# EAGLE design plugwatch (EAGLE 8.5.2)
AUTHOR: Noah Klugman; REV: B; TITLE: PlugWatch

## Sheet 1 of 4: Headers
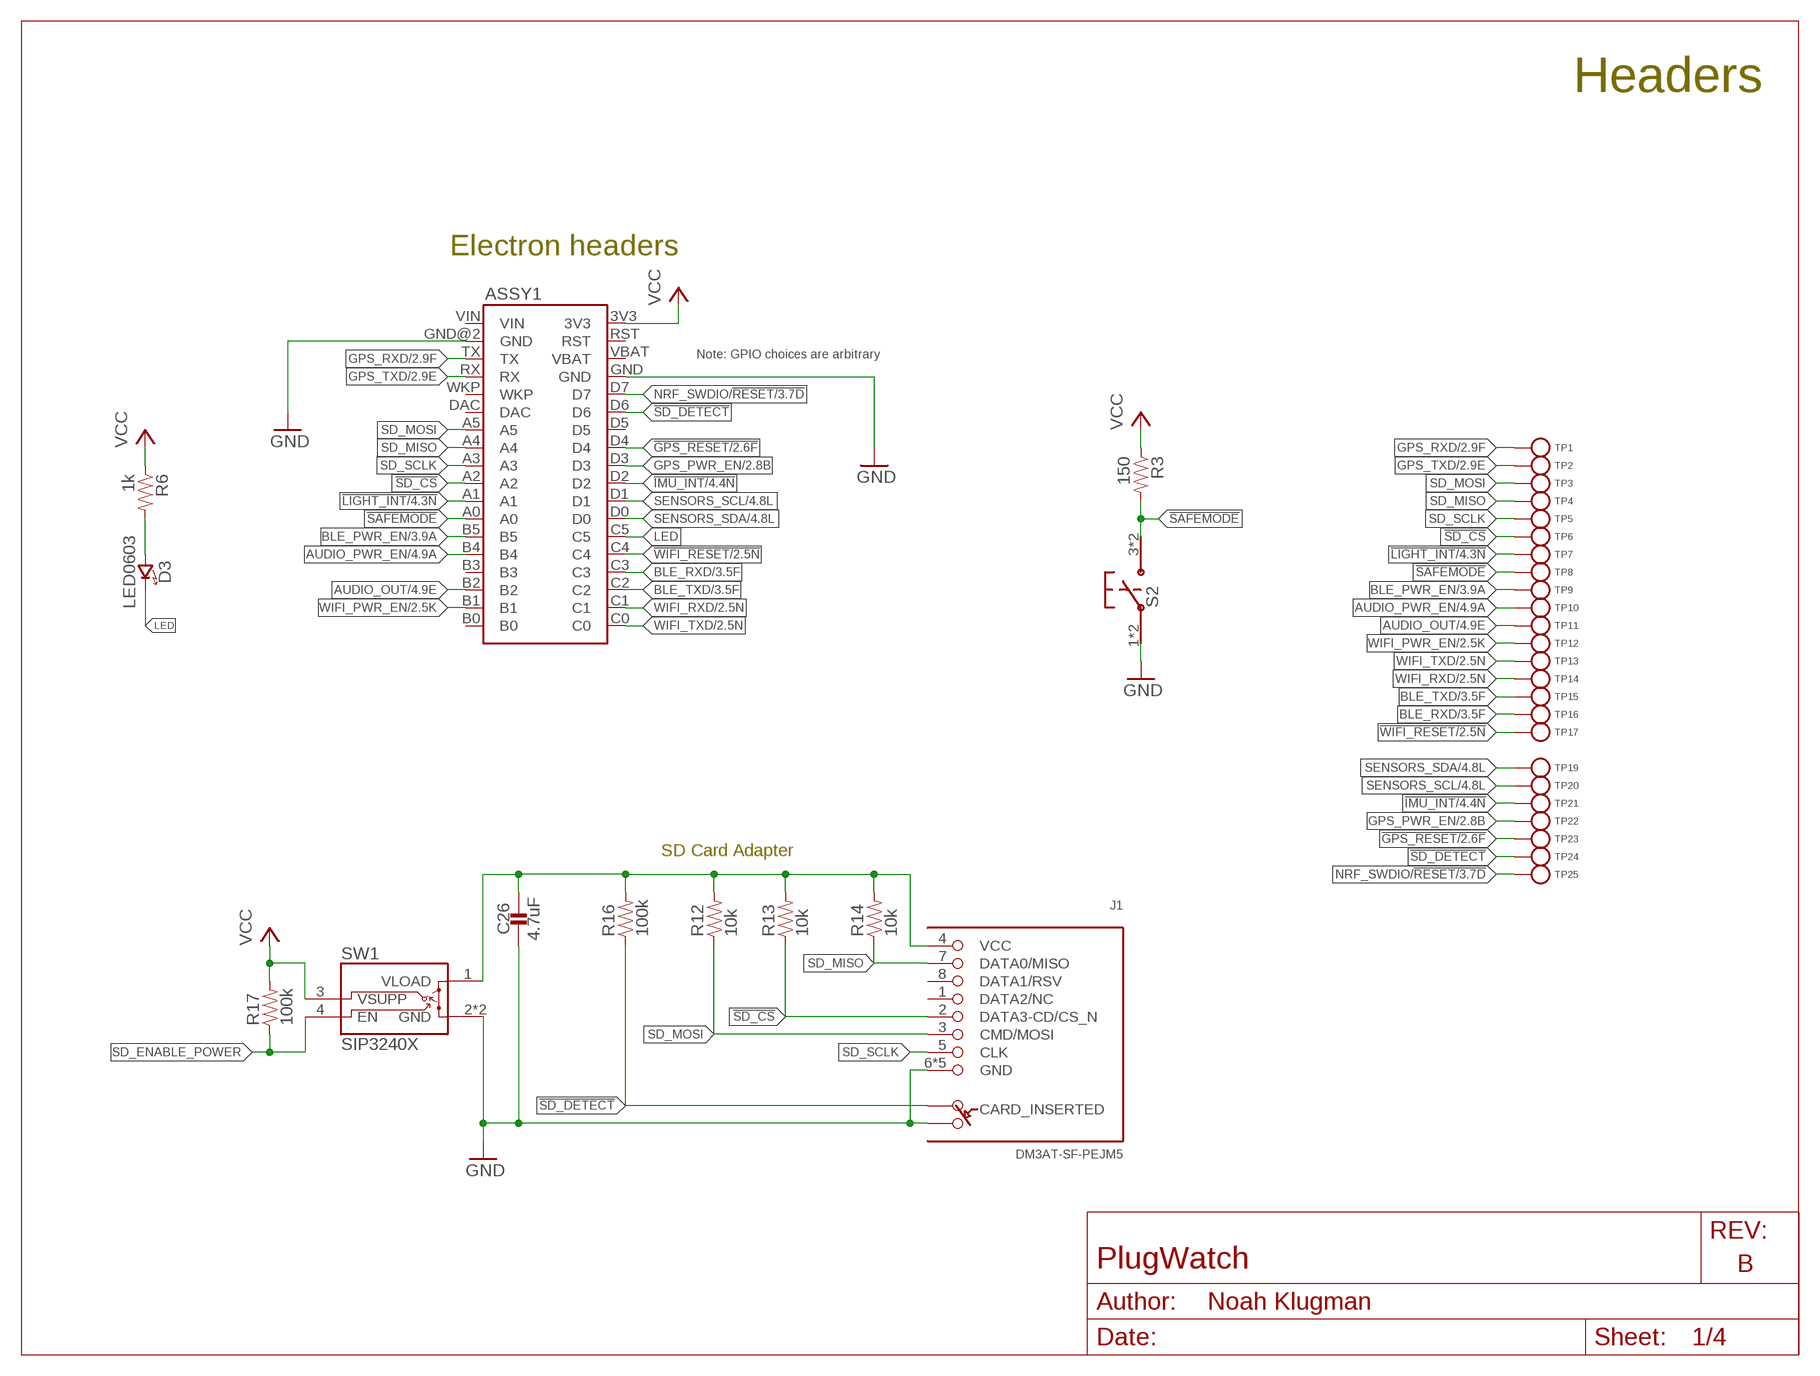
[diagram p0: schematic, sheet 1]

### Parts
ASSY1  ELECTRON  [ELECTRON_SINGLE-ROW]
C26  4.7uF  CAPACITOR0402_CAP  [0402_CAP]
D3  LED0603  [LED-0603]
J1  DM3AT-SF-PEJM5  [DM3AT-SF-PEJM5]
R3  150  RESISTOR0402_RES  [0402_RES]
R6  1k  RESISTOR0402_RES  [0402_RES]
R12  10k  RESISTOR0402_RES  [0402_RES]
R13  10k  RESISTOR0402_RES  [0402_RES]
R14  10k  RESISTOR0402_RES  [0402_RES]
R16  100k  RESISTOR0402_RES  [0402_RES]
R17  100k  RESISTOR0402_RES  [0402_RES]
S2  PTS645SM43SMTR92  [PTS645]
SW1  SIP3240X  [TDFN4]
TP1  TEST_POINT_0.040IN  [TESTPOINT_0.040IN]
TP2  TEST_POINT_0.040IN  [TESTPOINT_0.040IN]
TP3  TEST_POINT_0.040IN  [TESTPOINT_0.040IN]
TP4  TEST_POINT_0.040IN  [TESTPOINT_0.040IN]
TP5  TEST_POINT_0.040IN  [TESTPOINT_0.040IN]
TP6  TEST_POINT_0.040IN  [TESTPOINT_0.040IN]
TP7  TEST_POINT_0.040IN  [TESTPOINT_0.040IN]
TP8  TEST_POINT_0.040IN  [TESTPOINT_0.040IN]
TP9  TEST_POINT_0.040IN  [TESTPOINT_0.040IN]
TP10  TEST_POINT_0.040IN  [TESTPOINT_0.040IN]
TP11  TEST_POINT_0.040IN  [TESTPOINT_0.040IN]
TP12  TEST_POINT_0.040IN  [TESTPOINT_0.040IN]
TP13  TEST_POINT_0.040IN  [TESTPOINT_0.040IN]
TP14  TEST_POINT_0.040IN  [TESTPOINT_0.040IN]
TP15  TEST_POINT_0.040IN  [TESTPOINT_0.040IN]
TP16  TEST_POINT_0.040IN  [TESTPOINT_0.040IN]
TP17  TEST_POINT_0.040IN  [TESTPOINT_0.040IN]
TP19  TEST_POINT_0.040IN  [TESTPOINT_0.040IN]
TP20  TEST_POINT_0.040IN  [TESTPOINT_0.040IN]
TP21  TEST_POINT_0.040IN  [TESTPOINT_0.040IN]
TP22  TEST_POINT_0.040IN  [TESTPOINT_0.040IN]
TP23  TEST_POINT_0.040IN  [TESTPOINT_0.040IN]
TP24  TEST_POINT_0.040IN  [TESTPOINT_0.040IN]
TP25  TEST_POINT_0.040IN  [TESTPOINT_0.040IN]

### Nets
!GPS_RESET: ASSY1.D4 TP23.TESTPOINT ; also sheet 2
!IMU_INT: ASSY1.D2 TP21.TESTPOINT ; also sheet 4
!LIGHT_INT: ASSY1.A1 TP7.TESTPOINT ; also sheet 4
!SAFEMODE: ASSY1.A0 R3.2 S2.3 S2.4 TP8.TESTPOINT
!SD_CS: ASSY1.A2 J1.2(DATA3-CD/CS_N) R13.1 TP6.TESTPOINT
!SD_DETECT: ASSY1.D6 J1.A R16.1 TP24.TESTPOINT
!WIFI_RESET: ASSY1.C4 TP17.TESTPOINT ; also sheet 2
AUDIO_OUT: ASSY1.B2 TP11.TESTPOINT ; also sheet 4
AUDIO_PWR_EN: ASSY1.B4 TP10.TESTPOINT ; also sheet 4
BLE_PWR_EN: ASSY1.B5 TP9.TESTPOINT ; also sheet 3
BLE_RXD: ASSY1.C3 TP16.TESTPOINT ; also sheet 3
BLE_TXD: ASSY1.C2 TP15.TESTPOINT ; also sheet 3
GND: ASSY1.GND ASSY1.GND@2(GND) C26.2 J1.6(GND) J1.B J1.MOUNT0(GND) J1.MOUNT1(GND) J1.MOUNT2(GND) J1.MOUNT3(GND) S2.1 S2.2 SW1.2(GND) SW1.PAD(GND) ; also sheet 2,3,4
GPS_PWR_EN: ASSY1.D3 TP22.TESTPOINT ; also sheet 2
GPS_RXD: ASSY1.TX TP1.TESTPOINT ; also sheet 2
GPS_TXD: ASSY1.RX TP2.TESTPOINT ; also sheet 2
LED: ASSY1.C5 D3.C(CATHODE)
N$3: D3.A(ANODE) R6.2
N$18: C26.1 J1.4(VCC) R12.2 R13.2 R14.2 R16.2 SW1.1(VLOAD)
NRF_SWDIO/!RESET: ASSY1.D7 TP25.TESTPOINT ; also sheet 3
SD_ENABLE_POWER: R17.1 SW1.4(EN)
SD_MISO: ASSY1.A4 J1.7(DATA0/MISO) R14.1 TP4.TESTPOINT
SD_MOSI: ASSY1.A5 J1.3(CMD/MOSI) R12.1 TP3.TESTPOINT
SD_SCLK: ASSY1.A3 J1.5(CLK) TP5.TESTPOINT
SENSORS_SCL: ASSY1.D1 TP20.TESTPOINT ; also sheet 4
SENSORS_SDA: ASSY1.D0 TP19.TESTPOINT ; also sheet 4
VCC: ASSY1.3V3 R3.1 R6.1 R17.2 SW1.3(VSUPP) ; also sheet 2,3,4
WIFI_PWR_EN: ASSY1.B1 TP12.TESTPOINT ; also sheet 2
WIFI_RXD: ASSY1.C1 TP14.TESTPOINT ; also sheet 2
WIFI_TXD: ASSY1.C0 TP13.TESTPOINT ; also sheet 2
Unconnected: ASSY1.B0 ASSY1.B3 ASSY1.D5 ASSY1.DAC ASSY1.RST ASSY1.VBAT ASSY1.WKP J1.1(DATA2/NC) J1.8(DATA1/RSV)

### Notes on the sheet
- Headers
- Electron headers
- Note: GPIO choices are arbitrary
- SD Card Adapter

## Sheet 2 of 4: GPS and WiFi Radios
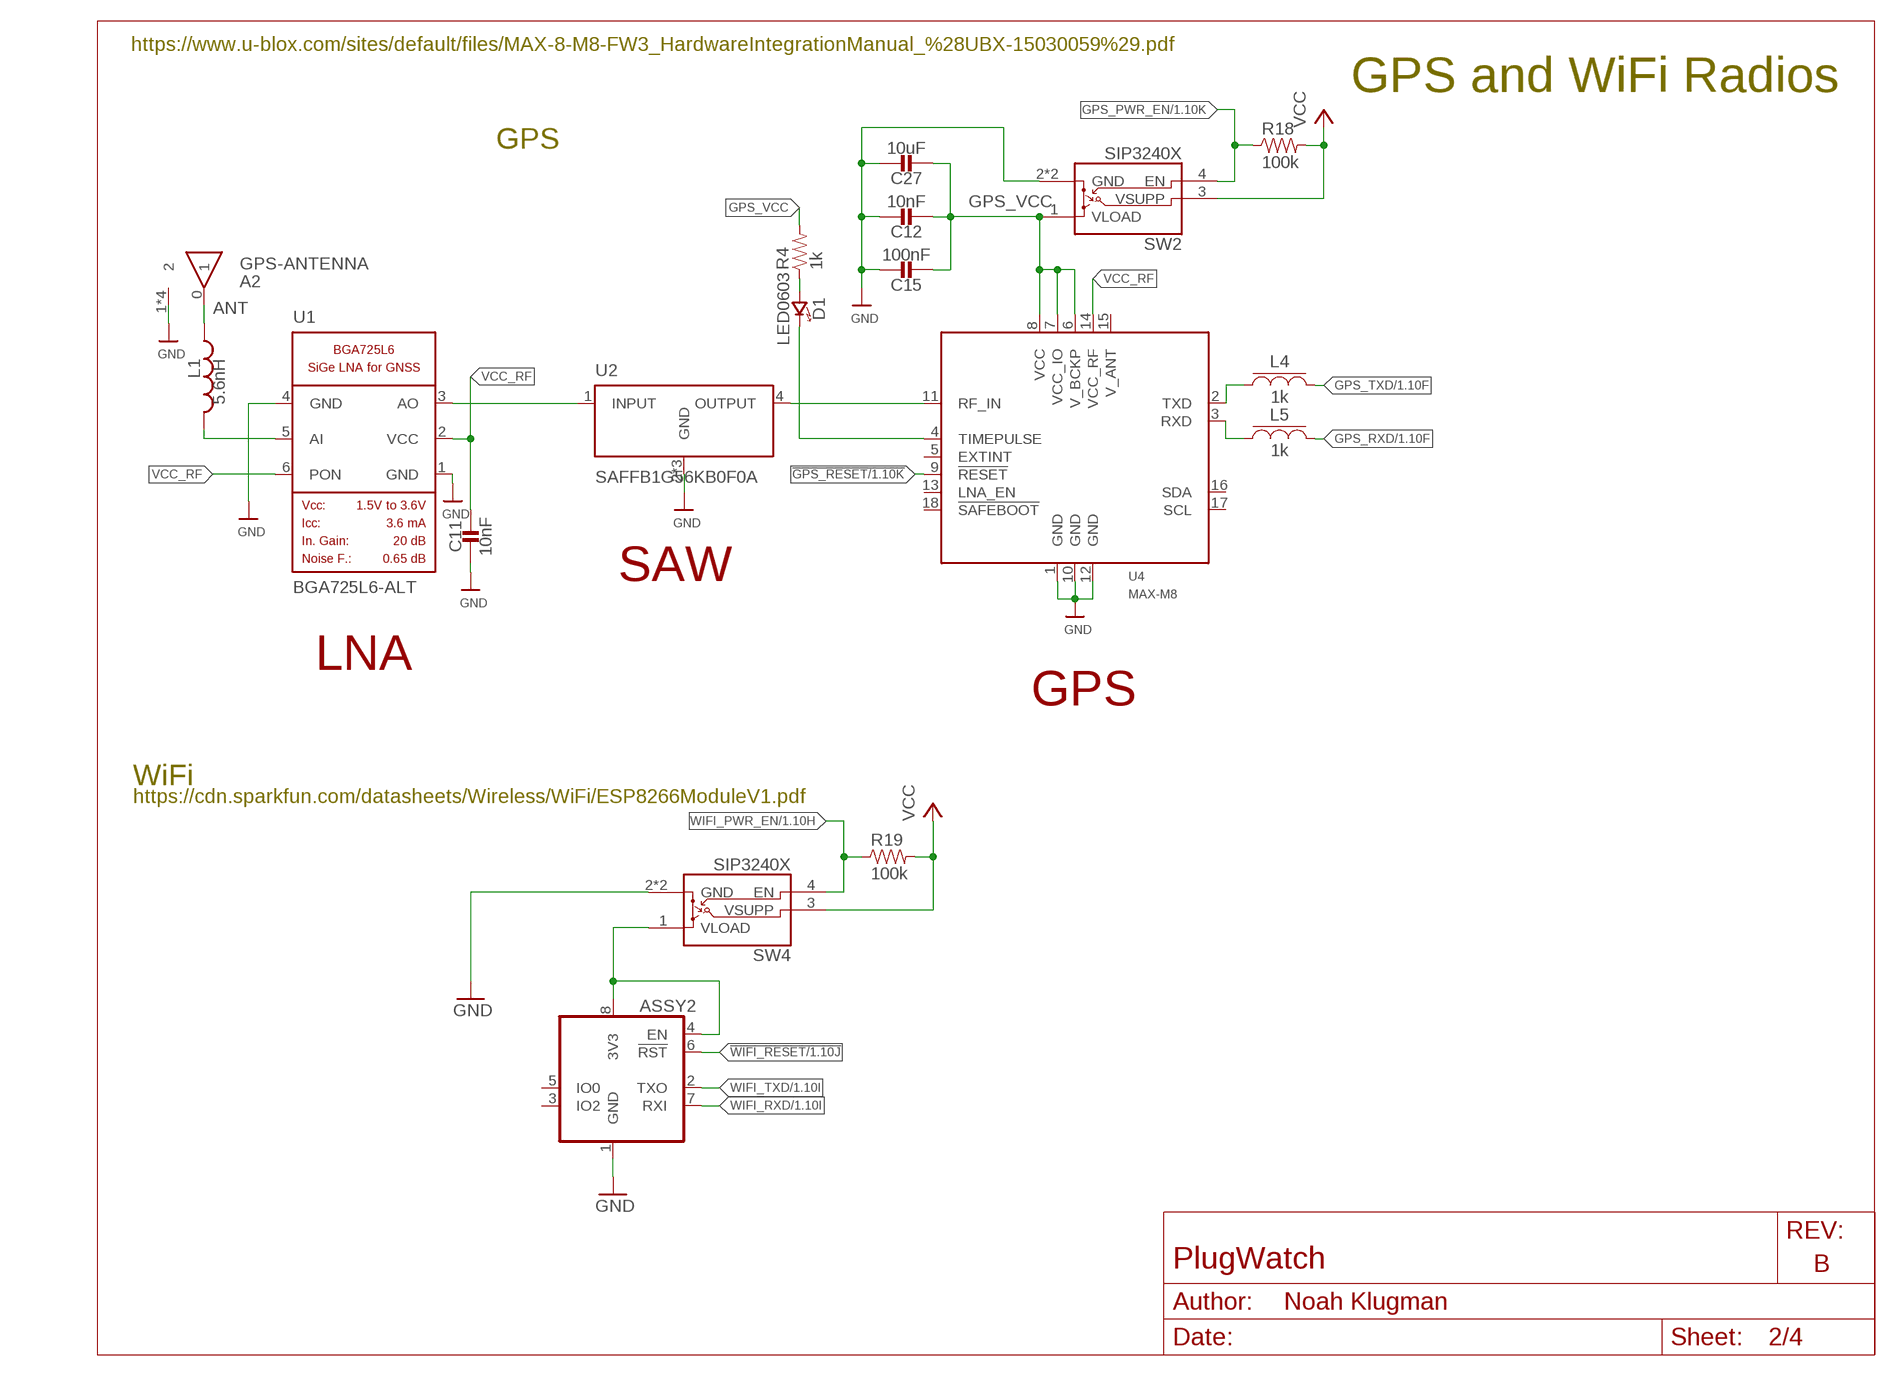
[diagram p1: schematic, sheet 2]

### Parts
A2  GPS-ANTENNA  [ANT1818B00BT1516S]
ASSY2  WRL-13678  [WRL-13678]
C11  10nF  CAPACITOR0402_CAP  [0402_CAP]
C12  10nF  CAPACITOR0402_CAP  [0402_CAP]
C15  100nF  CAPACITOR0402_CAP  [0402_CAP]
C27  10uF  CAPACITOR0402_CAP  [0402_CAP]
D1  LED0603  [LED-0603]
L1  5.6nH  INDUCTOR0402  [0402_CAP]
L4  1k  FERRITE_BEAD0402  [0402_CAP]
L5  1k  FERRITE_BEAD0402  [0402_CAP]
R4  1k  RESISTOR0402_RES  [0402_RES]
R18  100k  RESISTOR0402_RES  [0402_RES]
R19  100k  RESISTOR0402_RES  [0402_RES]
SW2  SIP3240X  [TDFN4]
SW4  SIP3240X  [TDFN4]
U1  BGA725L6-ALT  [LNA-TSLP-6-2-ALT]
U2  SAFFB1G56KB0F0A  FILTERS  [QCS5I]
U4  MAX-M8  [MAX-M8]

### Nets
!GPS_RESET: U4.9(!RESET) ; also sheet 1
!WIFI_RESET: ASSY2.6(!RST) ; also sheet 1
ANT: A2.0 L1.2
GND: A2.1 A2.2 A2.3 A2.4 ASSY2.1(GND) C11.1 C12.1 C15.1 C27.1 SW2.2(GND) SW2.PAD(GND) SW4.2(GND) SW4.PAD(GND) U1.1(GND) U1.4(GND) U2.2(GND) U2.3(GND) U2.5(GND) U4.1(GND) U4.10(GND) U4.12(GND) ; also sheet 1,3,4
GPS_PWR_EN: R18.1 SW2.4(EN) ; also sheet 1
GPS_RF_IN: U2.4(OUTPUT) U4.11(RF_IN)
GPS_RXD: L5.2 ; also sheet 1
GPS_TXD: L4.2 ; also sheet 1
GPS_VCC: C12.2 C15.2 C27.2 R4.2 SW2.1(VLOAD) U4.6(V_BCKP) U4.7(VCC_IO) U4.8(VCC)
LNA_IN: L1.1 U1.5(AI)
LNA_OUT: U1.3(AO) U2.1(INPUT)
N$1: D1.A(ANODE) R4.1
N$2: D1.C(CATHODE) U4.4(TIMEPULSE)
N$14: ASSY2.4(EN) ASSY2.8(3V3) SW4.1(VLOAD)
N$40: L4.1 U4.2(TXD)
N$41: L5.1 U4.3(RXD)
VCC: R18.2 R19.2 SW2.3(VSUPP) SW4.3(VSUPP) ; also sheet 1,3,4
VCC_RF: C11.2 U1.2(VCC) U1.6(PON) U4.14(VCC_RF)
WIFI_PWR_EN: R19.1 SW4.4(EN) ; also sheet 1
WIFI_RXD: ASSY2.7(RXI) ; also sheet 1
WIFI_TXD: ASSY2.2(TXO) ; also sheet 1
Unconnected: ASSY2.3(IO2) ASSY2.5(IO0) U4.5(EXTINT) U4.13(LNA_EN) U4.15(V_ANT) U4.16(SDA) U4.17(SCL) U4.18(!SAFEBOOT)

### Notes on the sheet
- https://www.u-blox.com/sites/default/files/MAX-8-M8-FW3_HardwareIntegrationManual_%28UBX-15030059%29.pdf
- GPS and WiFi Radios
- GPS
- SAW
- LNA
- GPS
- WiFi
- https://cdn.sparkfun.com/datasheets/Wireless/WiFi/ESP8266ModuleV1.pdf

## Sheet 3 of 4: BLE Radio
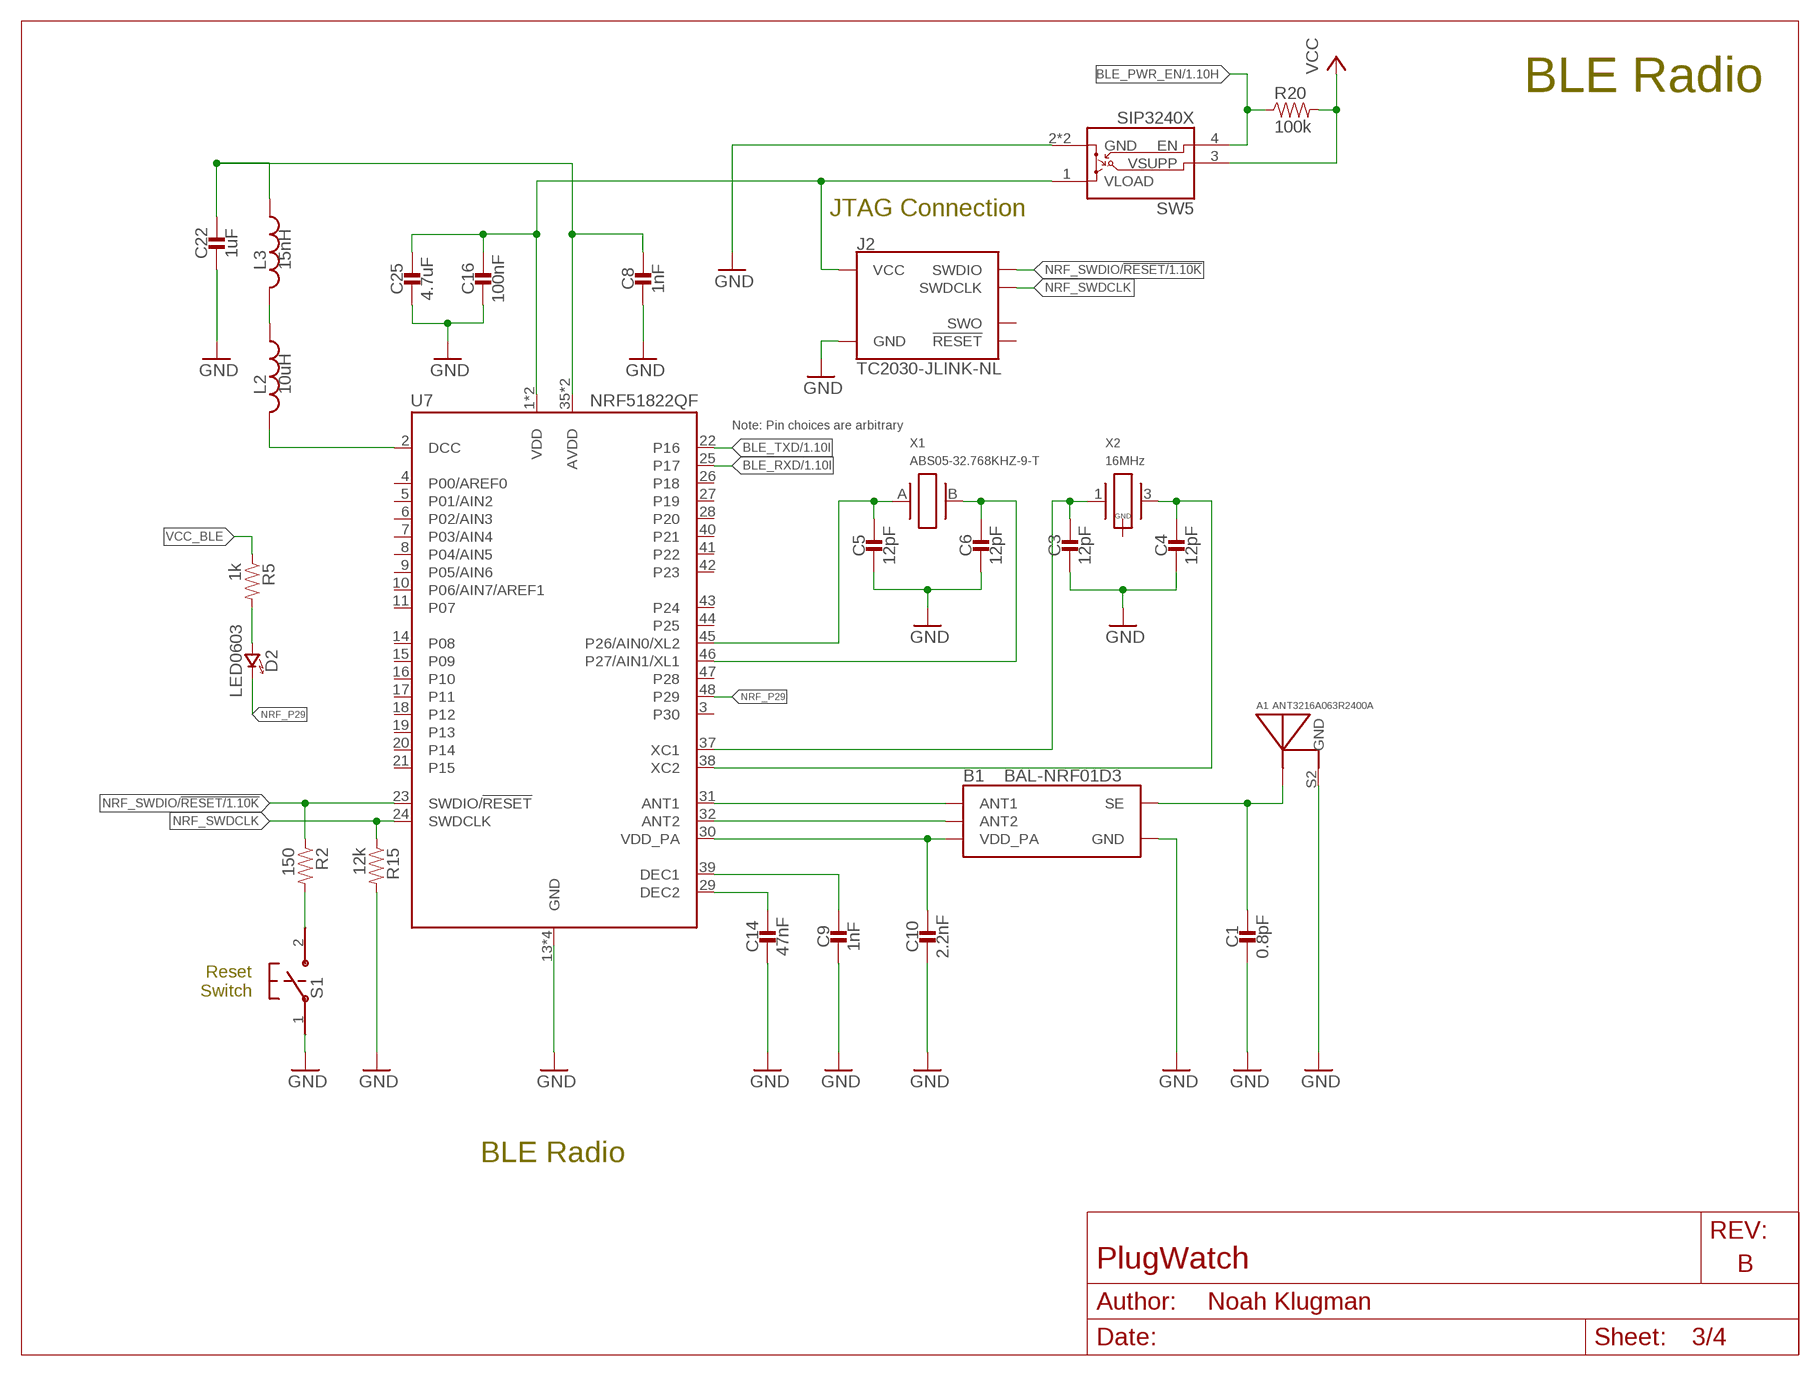
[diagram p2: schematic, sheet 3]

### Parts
A1  ANT3216A063R2400A  [ANT3216A063R2400A]
B1  BAL-NRF01D3  [BAL-NRF01D3]
C1  0.8pF  CAPACITOR0402_CAP  [0402_CAP]
C3  12pF  CAPACITOR0402_CAP  [0402_CAP]
C4  12pF  CAPACITOR0402_CAP  [0402_CAP]
C5  12pF  CAPACITOR0402_CAP  [0402_CAP]
C6  12pF  CAPACITOR0402_CAP  [0402_CAP]
C8  1nF  CAPACITOR0402_CAP  [0402_CAP]
C9  1nF  CAPACITOR0402_CAP  [0402_CAP]
C10  2.2nF  CAPACITOR0402_CAP  [0402_CAP]
C14  47nF  CAPACITOR0402_CAP  [0402_CAP]
C16  100nF  CAPACITOR0402_CAP  [0402_CAP]
C22  1uF  CAPACITOR0402_CAP  [0402_CAP]
C25  4.7uF  CAPACITOR0402_CAP  [0402_CAP]
D2  LED0603  [LED-0603]
J2  TC2030-JLINK-NL  [TC2030-IDC-NL]
L2  10uH  INDUCTOR0603  [0603_CAP]
L3  15nH  INDUCTOR0402  [0402_CAP]
R2  150  RESISTOR0402_RES  [0402_RES]
R5  1k  RESISTOR0402_RES  [0402_RES]
R15  12k  RESISTOR0402_RES  [0402_RES]
R20  100k  RESISTOR0402_RES  [0402_RES]
S1  B3U-1000P  [B3U-1000P]
SW5  SIP3240X  [TDFN4]
U7  NRF51822QF  [QFN-48-6MM]
X1  ABS05-32.768KHZ-9-T  [ABS05]
X2  16MHz  TXC-8Y  [TXC-8Y]

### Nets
AVDD1: C8.1 C22.1 L3.1 U7.35(AVDD) U7.36(AVDD)
BLE_PWR_EN: R20.1 SW5.4(EN) ; also sheet 1
BLE_RXD: U7.25(P17) ; also sheet 1
BLE_TXD: U7.22(P16) ; also sheet 1
DCC1: L2.2 U7.2(DCC)
GND: A1.S2(GND) B1.GND C1.2 C3.2 C4.2 C5.2 C6.2 C8.2 C9.2 C10.2 C14.2 C16.2 C22.2 C25.2 J2.5(GND) R15.2 S1.1 SW5.2(GND) SW5.PAD(GND) U7.13(GND) U7.33(GND) U7.34(GND) U7.GND ; also sheet 1,2,4
N$10: B1.ANT1 U7.31(ANT1)
N$12: B1.ANT2 U7.32(ANT2)
N$13: A1.S1(ANTENNA) B1.SE C1.1
N$15: L2.1 L3.2
N$20: C3.1 U7.37(XC1) X2.1
N$21: C4.1 U7.38(XC2) X2.3
N$22: C9.1 U7.39(DEC1)
N$24: C14.1 U7.29(DEC2)
N$25: D2.A(ANODE) R5.2
N$26: R2.2 S1.2
NRF_A2: C6.1 U7.46(P27/AIN1/XL1) X1.B
NRF_A3: C5.1 U7.45(P26/AIN0/XL2) X1.A
NRF_P29: D2.C(CATHODE) U7.48(P29)
NRF_SWDCLK: J2.4(SWDCLK) R15.1 U7.24(SWDCLK)
NRF_SWDIO/!RESET: J2.2(SWDIO) R2.1 U7.23(SWDIO/!RESET) ; also sheet 1
VCC: R20.2 SW5.3(VSUPP) ; also sheet 1,2,4
VCC_BLE: C16.1 C25.1 J2.1(VCC) R5.1 SW5.1(VLOAD) U7.1(VDD) U7.12(VDD)
VDD_PA1: B1.VCC(VDD_PA) C10.1 U7.30(VDD_PA)
Unconnected: J2.3(!RESET) J2.6(SWO) U7.3(P30) U7.4(P00/AREF0) U7.5(P01/AIN2) U7.6(P02/AIN3) U7.7(P03/AIN4) U7.8(P04/AIN5) U7.9(P05/AIN6) U7.10(P06/AIN7/AREF1) U7.11(P07) U7.14(P08) U7.15(P09) U7.16(P10) U7.17(P11) U7.18(P12) U7.19(P13) U7.20(P14) U7.21(P15) U7.26(P18) U7.27(P19) U7.28(P20) U7.40(P21) U7.41(P22) U7.42(P23) U7.43(P24) U7.44(P25) U7.47(P28) X2.2(GND) X2.4(GND)

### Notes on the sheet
- BLE Radio
- JTAG Connection
- Note: Pin choices are arbitrary
- Reset
  Switch
- BLE Radio

## Sheet 4 of 4: Sensors
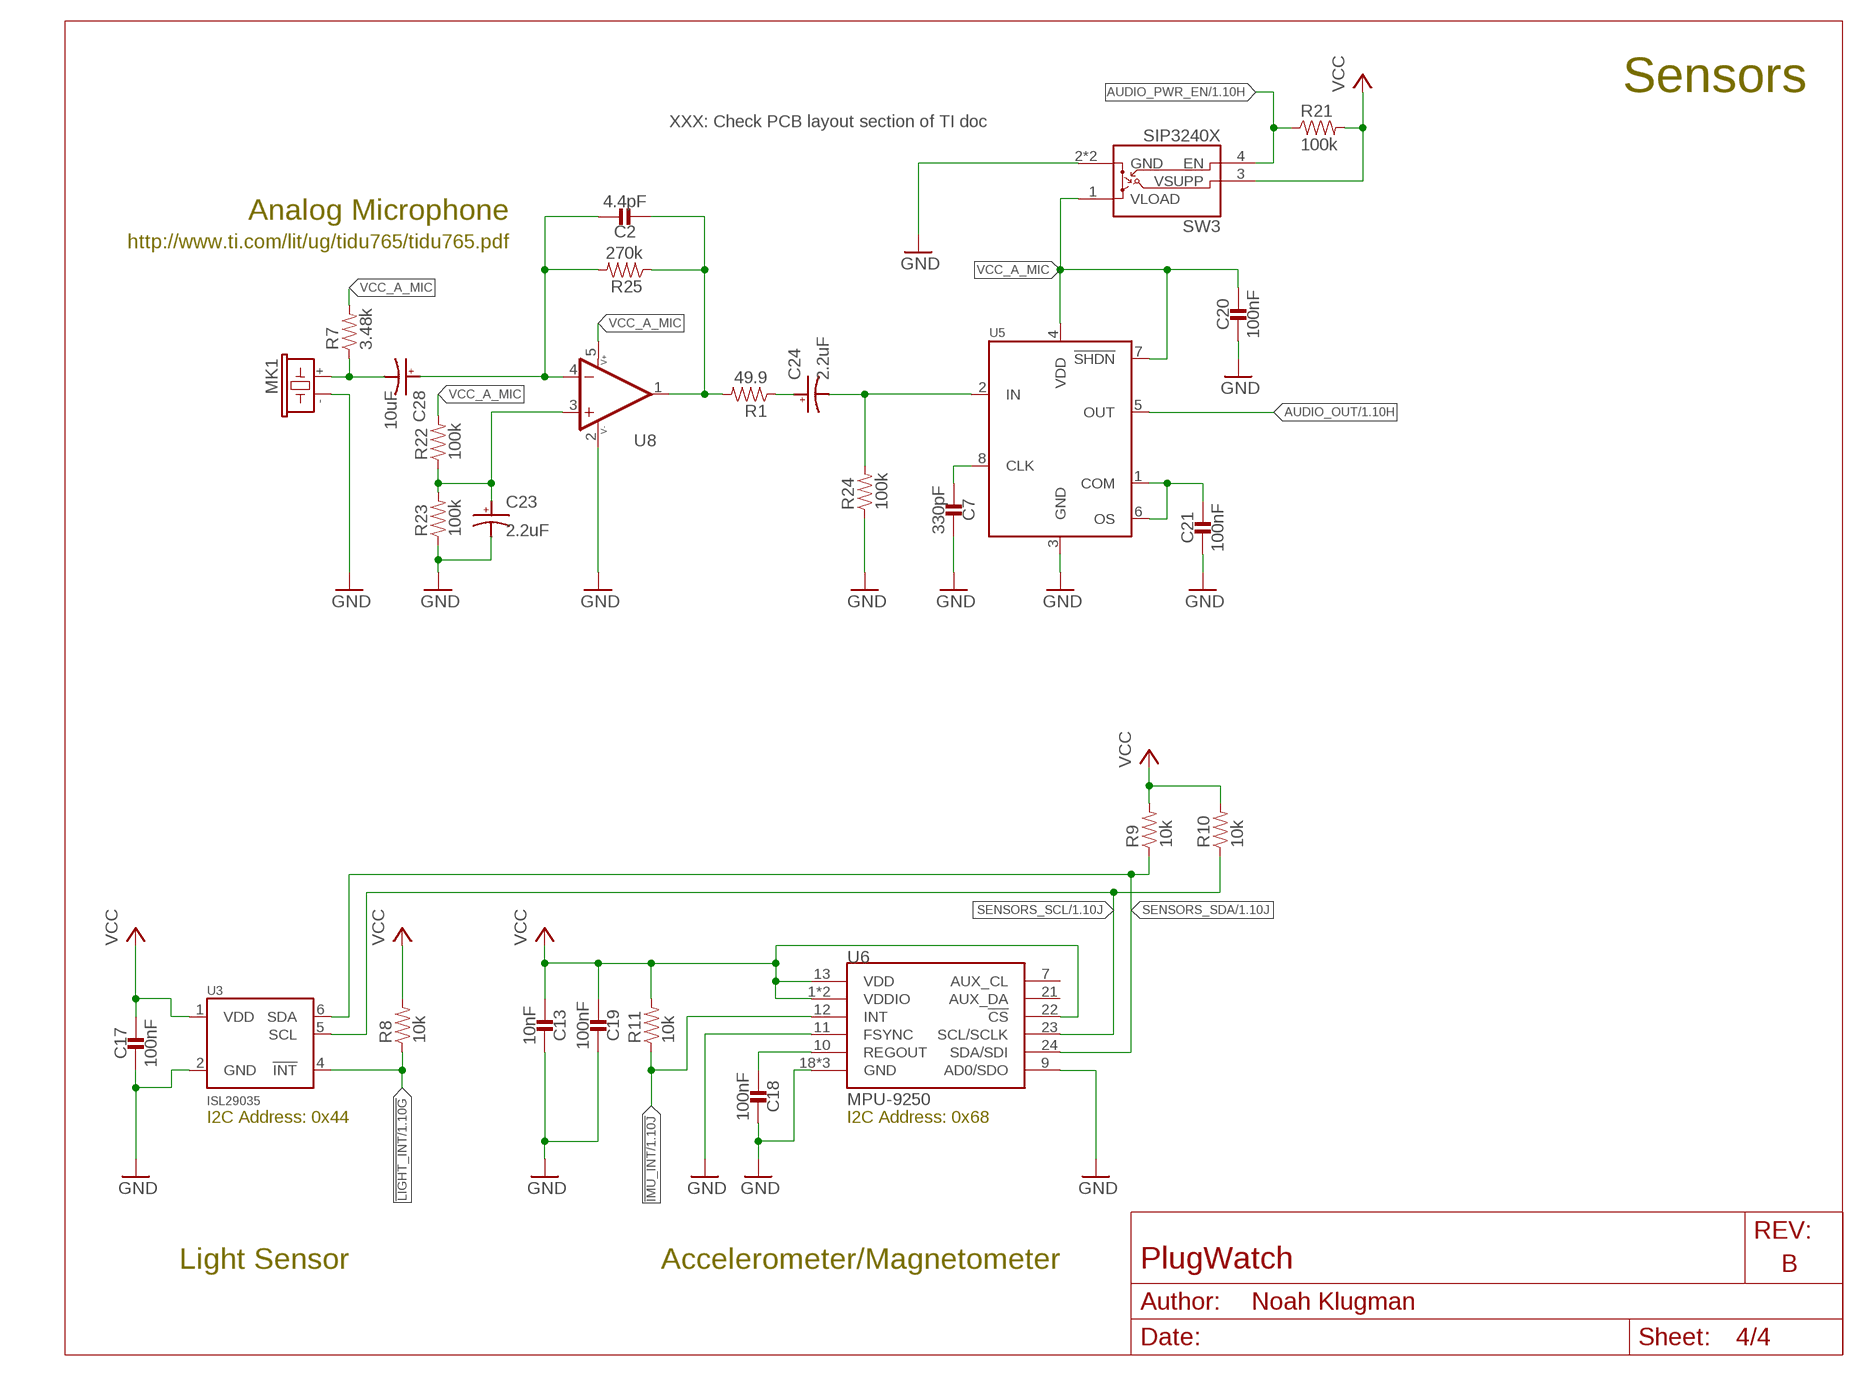
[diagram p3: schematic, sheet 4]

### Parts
C2  4.4pF  CAPACITOR0603_CAP  [0603_CAP]
C7  330pF  CAPACITOR0402_CAP  [0402_CAP]
C13  10nF  CAPACITOR0402_CAP  [0402_CAP]
C17  100nF  CAPACITOR0402_CAP  [0402_CAP]
C18  100nF  CAPACITOR0402_CAP  [0402_CAP]
C19  100nF  CAPACITOR0402_CAP  [0402_CAP]
C20  100nF  CAPACITOR0402_CAP  [0402_CAP]
C21  100nF  CAPACITOR0402_CAP  [0402_CAP]
C23  2.2uF  CAP_POL1206  [1206]
C24  2.2uF  CAP_POL1206  [1206]
C28  10uF  CAP_POL1206  [1206]
MK1  AOM-4546P-R  [MIC_AOM-4546P-R]
R1  49.9  RESISTOR0603_RES  [0603-RES]
R7  3.48k  RESISTOR0603_RES  [0603-RES]
R8  10k  RESISTOR0402_RES  [0402_RES]
R9  10k  RESISTOR0402_RES  [0402_RES]
R10  10k  RESISTOR0402_RES  [0402_RES]
R11  10k  RESISTOR0402_RES  [0402_RES]
R21  100k  RESISTOR0402_RES  [0402_RES]
R22  100k  RESISTOR0603_RES  [0603-RES]
R23  100k  RESISTOR0603_RES  [0603-RES]
R24  100k  RESISTOR0603_RES  [0603-RES]
R25  270k  RESISTOR0603_RES  [0603-RES]
SW3  SIP3240X  [TDFN4]
U3  ISL29035  [ODFN-6-1.5MMX1.6MM]
U5  MAX740XESA  [SOIC-8]
U6  MPU-9250  [QFN24_PAD]
U8  OPA322AIDBVT  [SOT23-5]

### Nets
!IMU_INT: R11.1 U6.12(INT) ; also sheet 1
!LIGHT_INT: R8.1 U3.4(!INT) ; also sheet 1
-AMP: C2.1 C28.2(CATHODE) R25.2 U8.4(-IN)
A_MIC_OUT: C24.1(ANODE) R24.2 U5.2(IN)
AUDIO_OUT: U5.5(OUT) ; also sheet 1
AUDIO_PWR_EN: R21.1 SW3.4(EN) ; also sheet 1
GND: C7.1 C13.2 C17.2 C18.2 C19.2 C20.2 C21.2 C23.1(ANODE) MK1.TERM- R23.1 R24.1 SW3.2(GND) SW3.PAD(GND) U3.2(GND) U5.3(GND) U6.9(AD0/SDO) U6.11(FSYNC) U6.18(GND) U6.20(GND) U6.CENTER(GND) U8.2(V-) ; also sheet 1,2,3
N$4: C28.1(ANODE) MK1.TERM+ R7.1
N$5: C2.2 R1.2 R25.1 U8.1(OUT)
N$6: C7.2 U5.8(CLK)
N$7: C24.2(CATHODE) R1.1
N$9: C23.2(CATHODE) R22.1 R23.2 U8.3(+IN)
N$11: C21.1 U5.1(COM) U5.6(OS)
REGOUT: C18.1 U6.10(REGOUT)
SENSORS_SCL: R10.1 U3.5(SCL) U6.23(SCL/SCLK) ; also sheet 1
SENSORS_SDA: R9.1 U3.6(SDA) U6.24(SDA/SDI) ; also sheet 1
VCC: C13.1 C17.1 C19.1 R8.2 R9.2 R10.2 R11.2 R21.2 SW3.3(VSUPP) U3.1(VDD) U6.1(VDDIO) U6.8(VDDIO) U6.13(VDD) U6.22(!CS) ; also sheet 1,2,3
VCC_A_MIC: C20.1 R7.2 R22.2 SW3.1(VLOAD) U5.4(VDD) U5.7(!SHDN) U8.5(V+)
Unconnected: U6.7(AUX_CL) U6.21(AUX_DA)

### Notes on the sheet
- Sensors
- XXX: Check PCB layout section of TI doc
- Analog Microphone
- http://www.ti.com/lit/ug/tidu765/tidu765.pdf
- I2C Address: 0x44 | I2C Address: 0x68
- Light Sensor | Accelerometer/Magnetometer

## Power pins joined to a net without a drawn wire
VIN: ASSY1.VIN

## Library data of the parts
A1 = chips:ANT3216A063R2400A: Yageo 2.4GHz; DIGIKEY: 311-1542-1-ND; MANUFACTURER: YAGEO; MPN: ANT3216A063R2400A
A2 = antenna:GPS-ANTENNA; DIGIKEY: 311-1531-ND
ASSY1 = electron:ELECTRON; DIGIKEY: S7051-ND,S7051-ND
ASSY2 = chips:WRL-13678: ESP8266 WiFi Module https://www.mouser.com/ds/2/813/ESP8266ModuleV1-1095236.pdf; DIGIKEY: 1568-1235-ND
B1 = chips:BAL-NRF01D3: 50 ohm nominal input / conjugate match balun to nRF51422-QFAA, nRF24LE1, nRF51822-QFAA/AB, with integrated harmonic filter; DIGIKEY: 497-13637-1-ND; MANUFACTURER: STMicroelectronics; MOUSER: 511-BAL-NRF01D3; MPN: BAL-NRF01D3
C1 = passives:CAPACITOR: 0402 Capacitor; DIGIKEY: 490-6269-1-ND
C2 = passives:CAPACITOR: 0402 Capacitor; DIGIKEY: 399-16187-1-ND
C3-C6 = passives:CAPACITOR: 0402 Capacitor; DIGIKEY: 490-6197-1-ND
C7 = passives:CAPACITOR: 0402 Capacitor; DIGIKEY: 490-6233-1-ND
C8 C9 = passives:CAPACITOR: 0402 Capacitor; DIGIKEY: 490-6366-1-ND
C10 = passives:CAPACITOR: 0402 Capacitor; DIGIKEY: 490-5419-1-ND
C11-C13 = passives:CAPACITOR: 0402 Capacitor; DIGIKEY: 490-7763-1-ND
C14 = passives:CAPACITOR: 0402 Capacitor; DIGIKEY: 490-11420-1-ND
C15-C21 = passives:CAPACITOR: 0402 Capacitor; DIGIKEY: 490-10777-1-ND
C22 = passives:CAPACITOR: 0402 Capacitor; DIGIKEY: 490-14457-1-ND
C23 C24 = passives:CAP_POL; DIGIKEY: 718-1131-1-ND
C25 C26 = passives:CAPACITOR: 0402 Capacitor; DIGIKEY: 445-5947-1-ND
C27 = passives:CAPACITOR: 0402 Capacitor; DIGIKEY: 490-8316-1-ND
C28 = passives:CAP_POL; DIGIKEY: 478-8481-1-ND
D1-D3 = leds:LED: LED; DIGIKEY: 160-1837-6-ND
J1 = connector:DM3AT-SF-PEJM5: CONN MICRO SD R/A PUSH-PUSH SMD; DIGIKEY: HR1964CT-ND
J2 = connector:TC2030-JLINK
L1 = passives:INDUCTOR: A very specific inductor; DIGIKEY: 490-11766-1-ND
L2 = passives:INDUCTOR: A very specific inductor; DIGIKEY: 490-4025-1-ND
L3 = passives:INDUCTOR: A very specific inductor; DIGIKEY: 587-1521-1-ND
L4 L5 = passives:FERRITE_BEAD; DIGIKEY: 490-4003-1-ND
MK1 = microphones:AOM-4546P-R: Electret microphone; DIGIKEY: 668-1224-ND
R1 = passives:RESISTOR: Resistor; DIGIKEY: 541-3003-1-ND
R2 R3 = passives:RESISTOR: Resistor; DIGIKEY: RMCF0402FT150RCT-ND
R4-R6 = passives:RESISTOR: Resistor; DIGIKEY: RMCF0402FT1K00CT-ND
R7 = passives:RESISTOR: Resistor; DIGIKEY: 541-3.48KHCT-ND
R8-R14 = passives:RESISTOR: Resistor; DIGIKEY: RMCF0402FT10K0CT-ND
R15 = passives:RESISTOR: Resistor; DIGIKEY: RMCF0402FT12K0CT-ND
R16-R21 = passives:RESISTOR: Resistor; DIGIKEY: 1276-3432-1-ND
R22-R24 = passives:RESISTOR: Resistor; DIGIKEY: 541-2972-1-ND
R25 = passives:RESISTOR: Resistor; DIGIKEY: 541-270KHCT-ND
S1 = switches:B3U: Switch; DIGIKEY: SW1020CT-ND; MANUFACTURER: Omron; MPN: B3U-1000P
S2 = switches:PTS645SM43SMTR92: Tactile Switch SPST-NO Top Actuated Surface Mount; DIGIKEY: CKN9112CT-ND
SW1-SW5 = signpost:SIP3240X: High power (2.4 A) high-side switch; DIGIKEY: SIP32402ADNP-T1GE4CT-ND
TP1-TP17 TP19-TP25 = headers:TEST_POINT_0.040IN: 0.040in Test Point; DIGIKEY: 5001K-ND
U1 = Particle:BGA725L6; DIGIKEY: BGA725L6E6327FTSA1CT-ND
U2 = Particle:FILTERS; ABACUS_TECHNOLOGIES: SAFFB1G56KB0F0A
U3 = chips:ISL29035: Optical Sensor Ambient 550nm I2C; DIGIKEY: ISL29035IROZ-T7CT-ND; MPN: ISL29035IROZ-T7
U4 = u-blox:MAX-M8; DIGIKEY: 672-1003-1-ND
U5 = chips:MAX740X; ROCHESTER_ELECTRONICS: MAX7405ESA
U6 = Testing:MPU-9250: NC pin 19. 2-6 & 14-17 not internally connected. May be used for PCB trace routing.; DIGIKEY: 1428-1019-1-ND; PROD_ID: IC-13192
U7 = chips:NRF51822: Multiprotocol Bluetooth® 4.0 low energy/2.4 GHz RF SoC; DIGIKEY: 1490-1049-1-ND; MANUFACTURER: Nordic Semi; MOUSER: 949-NRF51822-QFAC-R7; MPN: NRF51822-QFAC-R7
U8 = opamps:OPA322; DIGIKEY: 296-29511-1-ND
X1 = crystals:ABS05-32.768KHZ: 32.768kHz Crystal; DIGIKEY: 535-11897-1-ND
X2 = crystals:TXC-8Y: 2mmx1.6mm SMD Crystal; DIGIKEY: 887-2003-1-ND

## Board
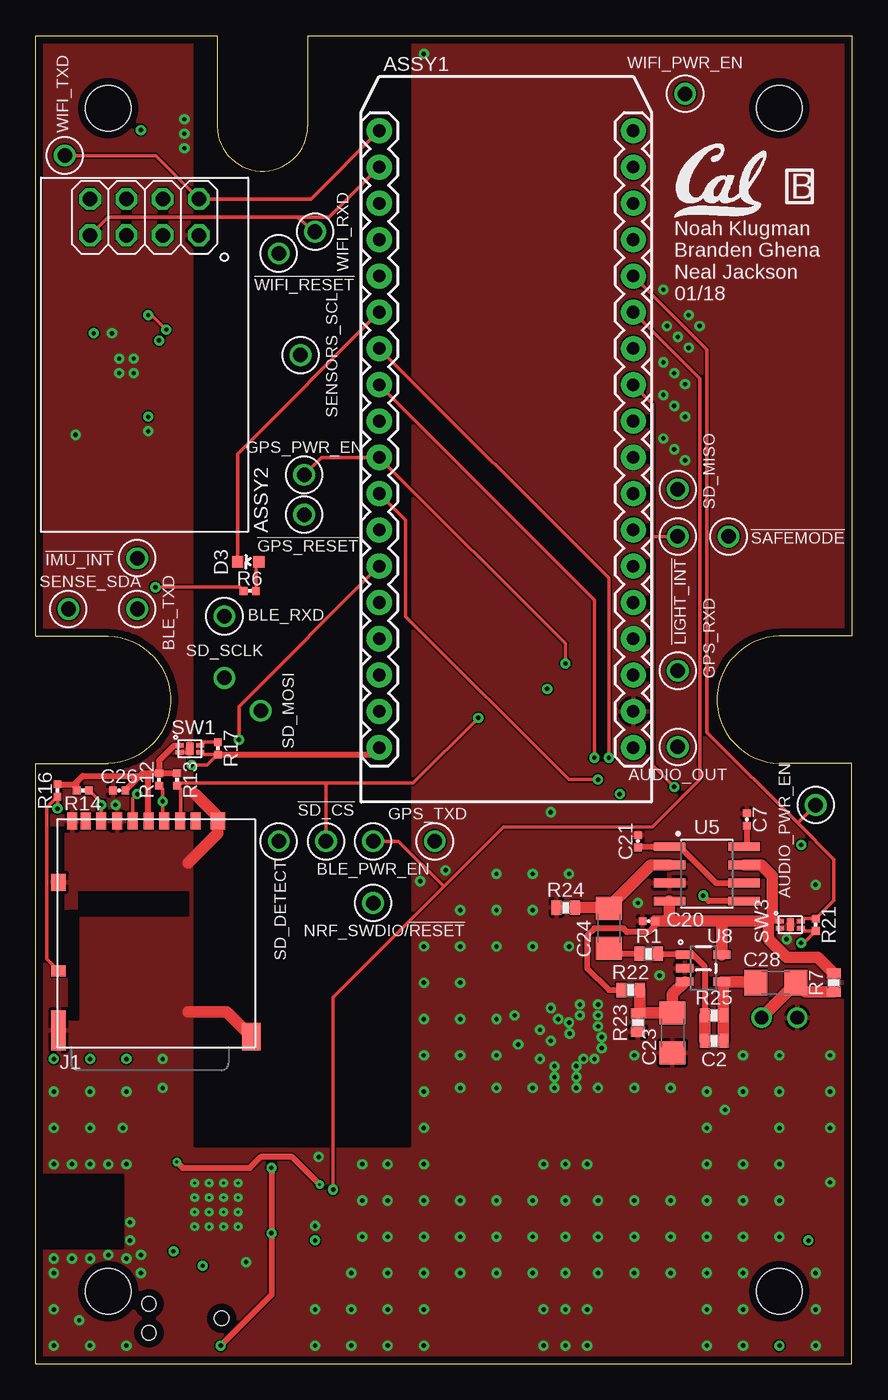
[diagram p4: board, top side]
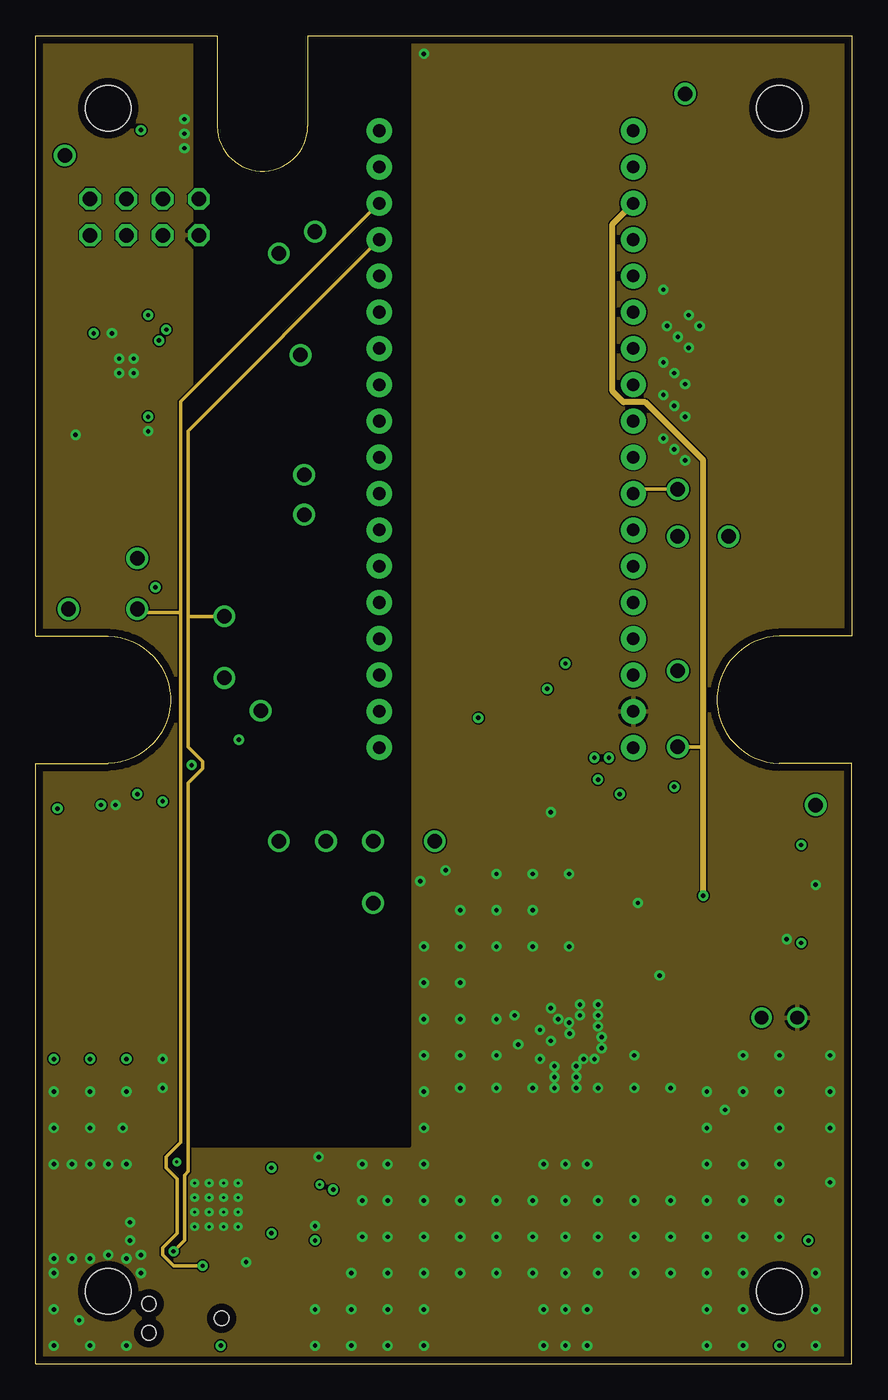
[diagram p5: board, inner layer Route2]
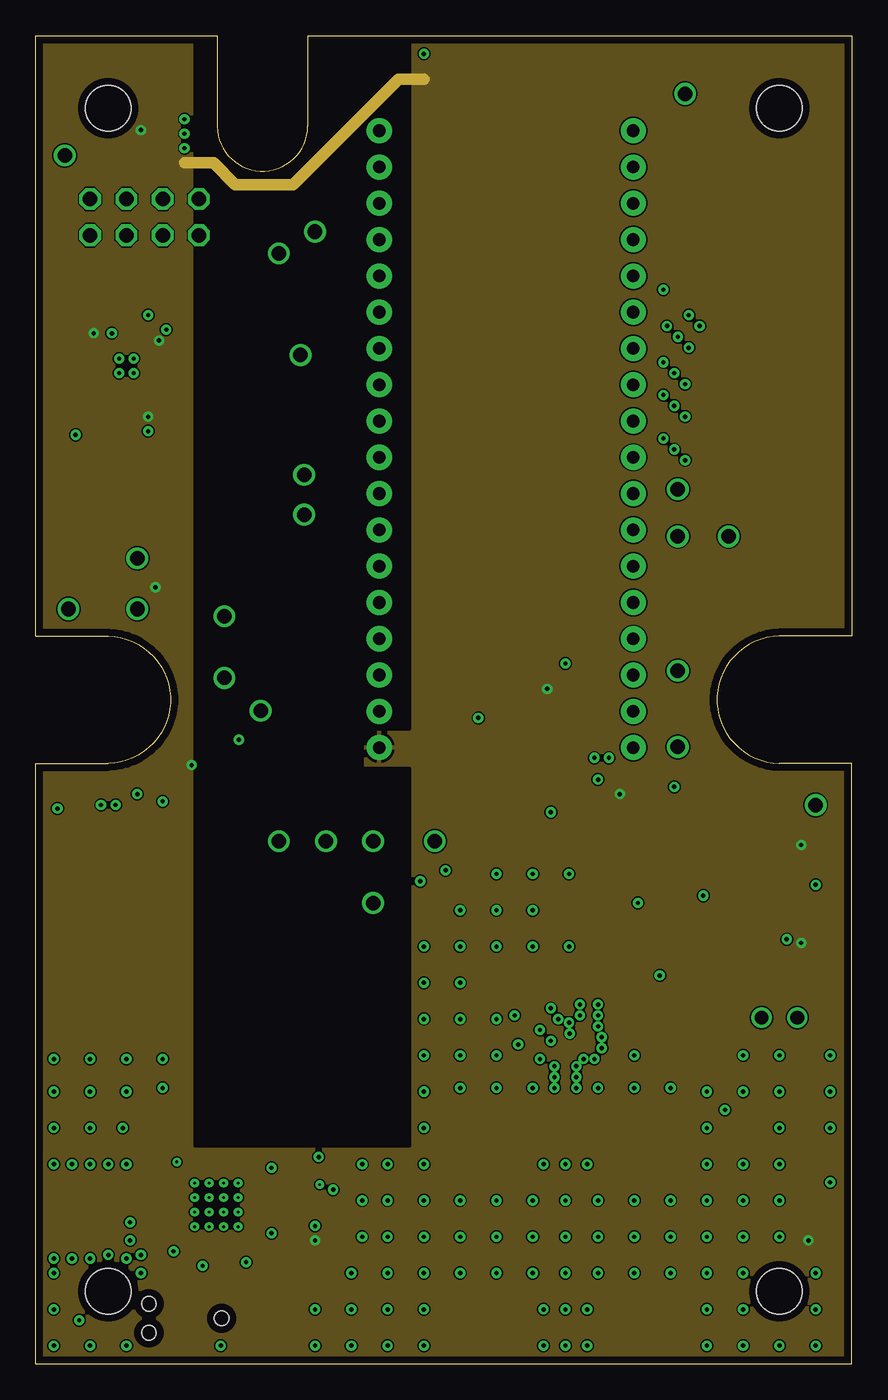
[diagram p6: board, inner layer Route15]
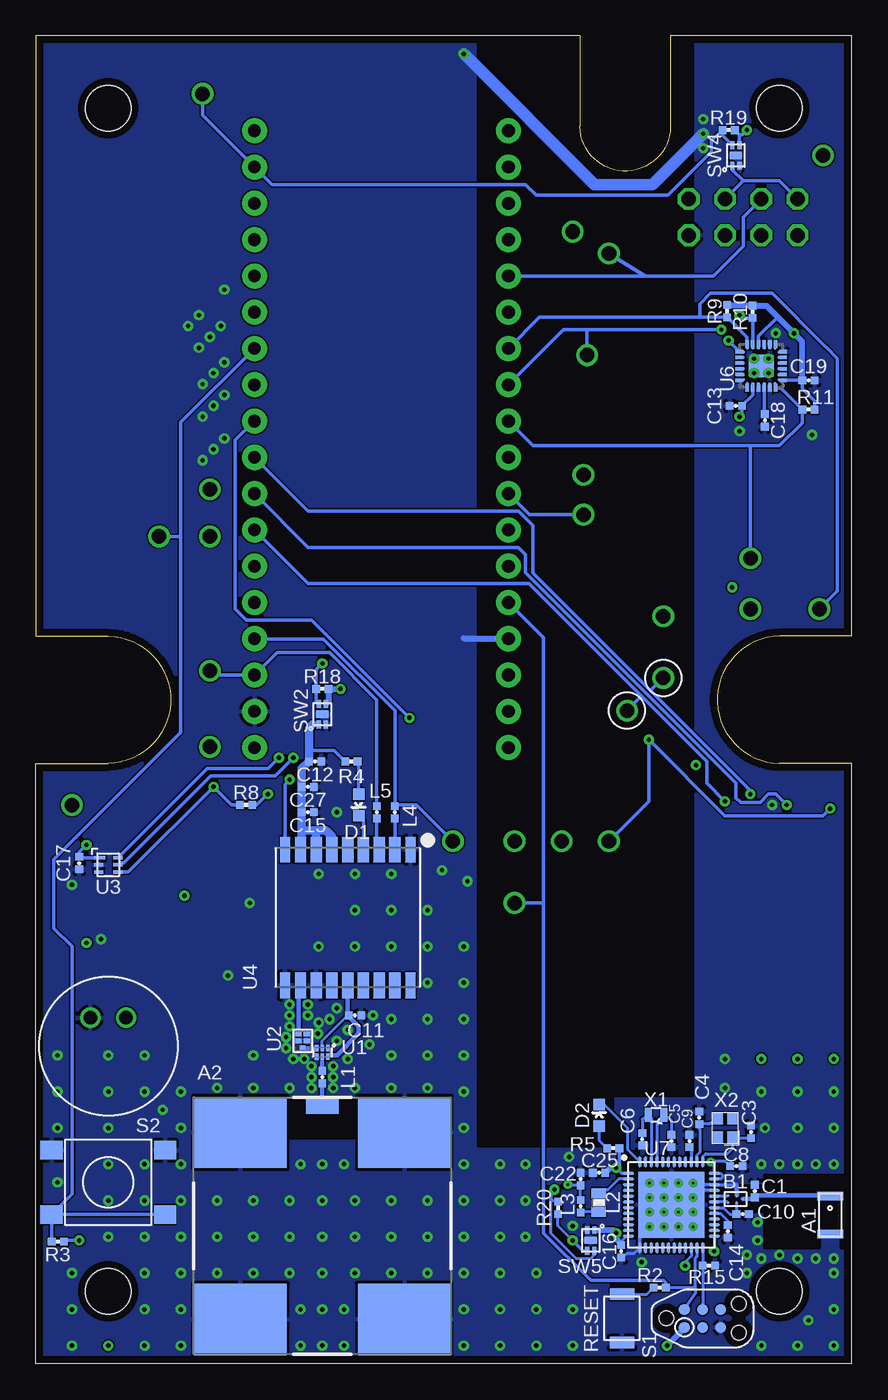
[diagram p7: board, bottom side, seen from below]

Size 57.15 x 92.96 mm. Coordinates in mm from the lower left corner, seen from the top.
Outline: 0,0 0,42.04 5.08,42.04 arc178 5.08,50.93 0,50.93 0,92.96 12.7,92.96 12.7,86.61 arc178 19.05,86.61 19.05,92.96 57.15,92.96 57.15,50.93 52.07,50.93 arc178 52.07,42.04 57.15,42.04 57.15,0 0,0
Copper layers (1+2*15+16): Top 0.0178mm / dielectric 12mil / Route2 0.0356mm / dielectric 28mil / Route15 0.0356mm / dielectric 12mil / Bottom 0.0178mm
Design rules "sunstone-4lyr_v1.0.0.3 *": minimum track width 4mil, minimum drill 8mil, track to track 4mil, track to pad 4mil, pad to pad 4mil, via to via 4mil, smd to smd 4mil, copper to edge 20mil, drill to drill 16mil, minimum pad ring 8mil, minimum via ring 8mil, stop-mask expansion 3mil, vias tented up to drill 50mil, thermal gap 8mil
Holes 3.17 mm at 5.08,87.88 52.07,87.88 5.08,5.08 52.07,5.08

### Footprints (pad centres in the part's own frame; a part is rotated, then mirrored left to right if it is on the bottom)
ANT3216A063R2400A = smd 0.6 x 1.8: S1 -1.325,0; S2 1.325,0
ANT1818B00BT1516S = smd 2.3 x 1.2: 0 0,-8.45 | smd 6.5 x 5: 1 -5.75,-6.55; 2 5.75,-6.55; 3 5.75,6.55; 4 -5.75,6.55
ELECTRON_SINGLE-ROW = drill 0.889 pad 1.753: 3V3 3.81,19.05; A0 31.75,1.27; A1 29.21,1.27; A2 26.67,1.27; A3 24.13,1.27; A4 21.59,1.27; A5 19.05,1.27; B0 46.99,1.27; B1 44.45,1.27; B2 41.91,1.27; B3 39.37,1.27; B4 36.83,1.27; B5 34.29,1.27; C0 46.99,19.05; C1 44.45,19.05; C2 41.91,19.05; C3 39.37,19.05; C4 36.83,19.05; C5 34.29,19.05; D0 31.75,19.05; D1 29.21,19.05; D2 26.67,19.05; D3 24.13,19.05; D4 21.59,19.05; D5 19.05,19.05; D6 16.51,19.05; D7 13.97,19.05; DAC 16.51,1.27; GND 11.43,19.05; GND@2 6.35,1.27; RST 6.35,19.05; RX 11.43,1.27; TX 8.89,1.27; VBAT 8.89,19.05; VIN 3.81,1.27; WKP 13.97,1.27
WRL-13678 = drill 1.016 octagon: 1 3.81,-1.27; 2 3.81,1.27; 3 1.27,-1.27; 4 1.27,1.27; 5 -1.27,-1.27; 6 -1.27,1.27; 7 -3.81,-1.27; 8 -3.81,1.27
BAL-NRF01D3 = smd 0.22 x 0.22: ANT1 -0.517,-0.25; ANT2 -0.517,0.25; GND 0.083,0.25; SE 0.516,0; VCC 0.083,-0.25
0402_CAP = smd 0.536 x 0.546: 1 -0.433,0; 2 0.433,0
0603_CAP = smd 0.7 x 1: 1 -0.65,0; 2 0.65,0
1206 = smd 1.6 x 1.8: 1 -1.4,0; 2 1.4,0
LED-0603 = smd 0.8 x 0.8: A 0,-0.75; C 0,0.75
DM3AT-SF-PEJM5 = smd 0.7 x 1.2: 1 3.2,-0.1; 2 2.1,-0.1; 3 1,-0.1; 4 -0.1,-0.1; 5 -1.2,-0.1; 6 -2.3,-0.1; 7 -3.4,-0.1; 8 -4.5,-0.1; B -5.45,-0.1 | smd 1 x 0.8: A -6.4,-10.6 | smd 1 x 1.2: MOUNT0 4.75,-0.1; MOUNT1 -6.4,-4.4 | smd 1 x 2.8: MOUNT2 -6.4,-14.75 | smd 1.3 x 1.9: MOUNT3 7.1,-15.2
TC2030-IDC-NL = smd 0.787 x 0.787: 1 -1.27,-0.635; 2 -1.27,0.635; 3 0,-0.635; 4 0,0.635; 5 1.27,-0.635; 6 1.27,0.635 | hole 1.016: -2.54,0; 2.54,1.016; 2.54,-1.016
MIC_AOM-4546P-R = drill 0.95: TERM+ 1.25,2; TERM- -1.25,2
0603-RES = smd 0.7 x 1: 1 -0.65,0; 2 0.65,0
0402_RES = smd 0.536 x 0.546: 1 -0.433,0; 2 0.433,0
B3U-1000P = smd 0.8 x 1.7: 1 -1.7,0; 2 1.7,0
PTS645 = smd 1.55 x 1.3: 1 -3.975,2.25; 2 3.975,2.25; 3 3.975,-2.25; 4 -3.975,-2.25
TDFN4 = smd 0.3 x 0.55: 1 -0.25,-0.725; 2 0.25,-0.725; 3 0.25,0.725; 4 -0.25,0.725 | smd 0.86 x 0.5: PAD 0,0
TESTPOINT_0.040IN = drill 1.016: TESTPOINT 0,0
LNA-TSLP-6-2-ALT = smd 0.45 x 0.25: 1 -0.3,0.4; 2 -0.3,0; 3 -0.3,-0.4; 4 0.3,-0.4; 5 0.3,0; 6 0.3,0.4
QCS5I = smd 0.35 x 0.425: 1 -0.5,0; 2 0,-0.287; 3 0.5,-0.287; 4 0.5,0.287; 5 0,0.287
ODFN-6-1.5MMX1.6MM = smd 0.8 x 0.25: 1 -0.6,0.5 | smd 0.65 x 0.25: 2 -0.675,0; 3 -0.675,-0.5; 4 0.675,-0.5; 5 0.675,0; 6 0.675,0.5
MAX-M8 = smd 1.8 x 0.7: 1 4.75,-4.4; 9 4.75,4.4; 10 -4.75,4.4; 18 -4.75,-4.4 | smd 1.8 x 0.8: 2 4.75,-3.3; 3 4.75,-2.2; 4 4.75,-1.1; 5 4.75,0; 6 4.75,1.1; 7 4.75,2.2; 8 4.75,3.3; 11 -4.75,3.3; 12 -4.75,2.2; 13 -4.75,1.1; 14 -4.75,0; 15 -4.75,-1.1; 16 -4.75,-2.2; 17 -4.75,-3.3
SOIC-8 = smd 0.61 x 2.21: 1 -1.905,-2.616; 2 -0.635,-2.616; 3 0.635,-2.616; 4 1.905,-2.616; 5 1.905,2.616; 6 0.635,2.616; 7 -0.635,2.616; 8 -1.905,2.616
QFN24_PAD = smd 0.5 x 0.25: 1 -1.55,1; 2 -1.55,0.6; 3 -1.55,0.2; 4 -1.55,-0.2; 5 -1.55,-0.6; 6 -1.55,-1; 13 1.55,-1; 14 1.55,-0.6; 15 1.55,-0.2; 16 1.55,0.2; 17 1.55,0.6; 18 1.55,1 | smd 0.08 x 0.13: 1$1 -1.32,1.06; 1$3 -1.26,0.94; P$33 1.26,-0.94; P$34 1.32,-1.06; P$58 1.26,0.94; P$59 1.32,1.06; P$68 -1.26,-0.94; P$69 -1.32,-1.06 | smd 0.1 x 0.185 rotated 45: 1$2 -1.25,1.024; P$49 1.024,-1.25 | smd 0.14 x 0.14: 1$4 -1.22,0.945; P$23 -0.945,-1.22; P$24 1.22,-0.945; P$36 0.945,1.22; P$51 0.945,-1.22; P$56 1.22,0.945; P$61 -0.945,1.22; P$66 -1.22,-0.945 | smd 0.05 x 0.05: 1$5 -1.175,0.97; P$25 -0.97,-1.175; P$31 1.175,-0.97; P$37 0.97,1.175; P$52 0.97,-1.175; P$57 1.175,0.97; P$62 -0.97,1.175; P$67 -1.175,-0.97 | smd 0.25 x 0.5: 7 -1,-1.55; 8 -0.6,-1.55; 9 -0.2,-1.55; 10 0.2,-1.55; 11 0.6,-1.55; 12 1,-1.55; 19 1,1.55; 20 0.6,1.55; 21 0.2,1.55; 22 -0.2,1.55; 23 -0.6,1.55; 24 -1,1.55 | smd 0.25 x 0.25: CENTER 0,0 | smd 0.4 x 0.4: DBBADFE -0.675,0.24 | smd 0.6 x 1.2: DBBADFE1 -0.575,-0.195 | smd 0.25 x 0.3: P$1 -0.2,1.3; P$3 0.2,1.3; P$5 0.6,1.3; P$11 -0.6,1.3; P$16 0.2,-1.3; P$18 -0.2,-1.3; P$20 -0.6,-1.3; P$26 0.6,-1.3 | smd 0.3 x 0.25: P$2 -1.3,0.2; P$4 -1.3,0.6; P$28 -1.3,-0.2; P$38 -1.3,-0.6; P$40 1.3,0.2; P$42 1.3,-0.2; P$44 1.3,-0.6; P$50 1.3,0.6 | smd 0.1 x 0.185 rotated 225: P$7 1.25,-1.024; P$60 -1.024,1.25 | smd 1.1 x 1.59: P$13 0.325,0 | smd 0.3 x 0.5 rotated 315: P$14 -0.592,0.512 | smd 0.5 x 1.59: P$15 -0.27,0 | smd 0.1 x 0.185 rotated 135: P$22 -1.024,-1.25; P$55 1.25,1.024 | smd 0.13 x 0.08: P$27 -0.94,-1.26; P$29 -1.06,-1.32; P$39 0.94,1.26; P$41 1.06,1.32; P$53 0.94,-1.26; P$54 1.06,-1.32; P$63 -0.94,1.26; P$64 -1.06,1.32 | smd 0.1 x 0.185 rotated 315: P$35 1.024,1.25; P$65 -1.25,-1.024
QFN-48-6MM = smd 0.8 x 0.203: 1 -3,2.2; 2 -3,1.8; 3 -3,1.4; 4 -3,1; 5 -3,0.6; 6 -3,0.2; 7 -3,-0.2; 8 -3,-0.6; 9 -3,-1; 10 -3,-1.4; 11 -3,-1.8; 12 -3,-2.2; 25 3,-2.2; 26 3,-1.8; 27 3,-1.4; 28 3,-1; 29 3,-0.6; 30 3,-0.2; 31 3,0.2; 32 3,0.6; 33 3,1; 34 3,1.4; 35 3,1.8; 36 3,2.2 | smd 0.203 x 0.8: 13 -2.2,-3; 14 -1.8,-3; 15 -1.4,-3; 16 -1,-3; 17 -0.6,-3; 18 -0.2,-3; 19 0.2,-3; 20 0.6,-3; 21 1,-3; 22 1.4,-3; 23 1.8,-3; 24 2.2,-3; 37 2.2,3; 38 1.8,3; 39 1.4,3; 40 1,3; 41 0.6,3; 42 0.2,3; 43 -0.2,3; 44 -0.6,3; 45 -1,3; 46 -1.4,3; 47 -1.8,3; 48 -2.2,3 | smd 4.6 x 4.6: GND 0,0
SOT23-5 = smd 0.6 x 1.2: 1 -0.95,-1.3; 2 0,-1.3; 3 0.95,-1.3; 4 0.95,1.3; 5 -0.95,1.3
ABS05 = smd 0.5 x 1: A -0.55,0; B 0.55,0
TXC-8Y = smd 0.8 x 0.7: 1 -0.65,-0.5; 2 0.65,-0.5; 3 0.65,0.5; 4 -0.65,0.5

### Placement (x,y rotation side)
A1  1.52,10.41 270 bottom
A2  37.08,9.65 180 bottom
ASSY1  43.1,39.32 90 top
ASSY2  7.62,80.26 0 top
B1  8.15,11.53 0 bottom
C1  6.8,12.09 90 bottom
C2  47.5,22.61 180 top
C3  7.06,16.23 90 bottom
C4  10.69,17.22 90 bottom
C5  12.65,15.6 270 bottom
C6  14.68,15.72 270 bottom
C7  49.78,38.1 270 top
C8  8.09,13.84 0 bottom
C9  11.38,15.6 90 bottom
C10  7.66,10.47 0 bottom
C11  34.8,24.38 180 bottom
C12  37.59,42.16 180 bottom
C13  8.13,67.06 180 bottom
C14  8.69,9.27 270 bottom
C15  38.1,38.61 180 bottom
C16  16.16,7.87 270 bottom
C17  54.1,35.05 270 bottom
C18  6.1,66.04 270 bottom
C19  3.05,68.83 0 bottom
C20  42.93,30.99 180 top
C21  42.16,36.58 90 top
C22  19,12.93 90 bottom
C23  44.58,23.16 90 top
C24  40.13,30.48 270 top
C25  17.7,13.37 180 bottom
C26  5.84,40.13 180 top
C27  38.1,40.39 180 bottom
C28  51.82,26.67 180 top
D1  34.54,39.12 180 bottom
D2  17.7,17.4 0 bottom
D3  14.88,56.13 90 top
J1  8,38.1 0 top
J2  10.46,3.17 0 bottom
L1  37.08,20.07 270 bottom
L2  17.73,11.28 90 bottom
L3  19,11.02 270 bottom
L4  32,38.61 90 bottom
L5  33.27,38.61 90 bottom
MK1  52.07,22.23 0 bottom
R1  42.93,28.7 0 top
R2  13.46,5.34 180 bottom
R3  55.6,8.56 180 bottom
R4  35.05,42.16 180 bottom
R5  16.71,15.09 180 bottom
R6  14.99,54.1 0 top
R7  55.88,26.67 90 top
R8  42.42,39.12 0 bottom
R9  8.74,73.69 90 bottom
R10  6.96,73.63 90 bottom
R11  3.05,66.8 0 bottom
R12  8.64,40.89 90 top
R13  9.91,40.89 90 top
R14  3.3,40.13 180 top
R15  10.02,6.87 0 bottom
R16  1.52,40.13 90 top
R17  12.75,43.08 270 top
R18  37.08,47.24 0 bottom
R19  8.64,86.36 0 bottom
R20  20.57,10.92 270 bottom
R21  54.61,30.73 270 top
R22  41.66,26.16 180 top
R23  42.16,23.88 90 top
R24  37.11,31.93 0 top
R25  47.5,24.38 0 top
S1  16.1,3.17 90 bottom
S2  52.07,12.7 0 bottom
SW1  10.79,43.05 270 top
SW2  37.08,45.47 0 bottom
SW3  52.83,30.73 270 top
SW4  8.13,84.58 0 bottom
SW5  18.29,8.64 180 bottom
TP1  44.96,48.51 0 top
TP2  27.94,36.58 0 top
TP3  15.75,45.72 0 bottom
TP4  44.96,61.21 0 top
TP5  13.21,48.01 0 bottom
TP6  20.32,36.58 0 top
TP7  44.96,57.91 0 top
TP8  48.51,57.91 0 top
TP9  23.62,36.58 0 top
TP10  54.61,39.12 0 top
TP11  44.96,43.18 0 top
TP12  45.47,88.9 0 top
TP13  2.03,84.58 0 top
TP14  19.56,79.25 0 top
TP15  7.11,52.83 0 top
TP16  13.21,52.32 0 top
TP17  17.02,77.72 0 top
TP19  2.29,52.83 0 top
TP20  18.54,70.61 0 top
TP21  7.11,56.39 0 top
TP22  18.8,62.23 0 top
TP23  18.8,59.44 0 top
TP24  17.02,36.58 0 top
TP25  23.62,32.26 0 top
U1  37.08,21.79 270 bottom
U2  38.46,22.61 90 bottom
U3  52.07,34.92 0 bottom
U4  35.31,31.24 90 bottom
U5  46.99,34.29 270 top
U6  6.35,69.85 0 bottom
U7  12.65,11.13 0 bottom
U8  46.74,27.69 270 top
U$3  [UCB_CAL_200MIL]  44.7,80.26 0 top
X1  13.72,17.42 180 bottom
X2  8.89,16.51 90 bottom

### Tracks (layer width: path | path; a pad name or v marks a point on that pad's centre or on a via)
!GPS_RESET  (via drill 0.3)
  Top 0.254: v39.37,40.89 37.34,40.89 25.91,52.32 25.91,59.05 ASSY1.D4
  Bottom 0.254: v39.37,40.89 39.71,40.56 U4.9 | TP23.TESTPOINT 22.58,59.44 ASSY1.D4
!IMU_INT
  Bottom 0.254: U6.12 4.98,68.3 R11.1 3.48,65.86 5.08,64.26 7.11,64.26 | 7.11,64.26 22.33,64.26 ASSY1.D2 | TP21.TESTPOINT 7.11,64.26
!LIGHT_INT  (via drill 0.3)
  Top 0.254: ASSY1.A1 43.18,67.18 43.18,57.91 | v44.7,40.39 43.18,41.91 43.18,57.91 | TP7.TESTPOINT 43.18,57.91
  Bottom 0.254: U3.4 50.66,34.42 v44.7,40.39 43.43,39.12 R8.1
!SAFEMODE
  Bottom 0.254: R3.2 56.05,8.57 S2.4 | S2.3 S2.4 | S2.4 54.61,11.88 54.61,29.21 55.88,30.48 55.88,35.31 46.99,44.2 46.99,57.91 | ASSY1.A0 46.99,65.91 46.99,57.91 | TP8.TESTPOINT 46.99,57.91
!SD_CS  (via drill 0.3)
  Top 0.254: J1.2 10.16,38.06 10.16,40.21 R13.1 10.09,40.64 20.32,40.64 | 20.32,40.64 26.42,40.64 v30.99,45.21 | TP6.TESTPOINT 20.32,40.64
  Bottom 0.254: v30.99,45.21 37.85,52.07 42.42,52.07 43.18,52.83 43.18,64.64 ASSY1.A2
!SD_DETECT  (via drill 0.3)
  Top 0.254: J1.A 0.76,28.34 0.76,38.94 R16.1 v1.52,38.86 | v14.22,43.69 14.22,46 ASSY1.D6
  Bottom 0.254: v1.52,38.86 2.03,38.35 8.89,38.35 v14.22,43.69 14.22,39.88 14.22,39.37 TP24.TESTPOINT
!WIFI_RESET
  Bottom 0.254: ASSY1.C4 14.48,76.15 | 14.48,76.15 9.7,76.15 7.62,78.23 7.62,80.26 ASSY2.6 | TP17.TESTPOINT 14.48,76.15
-AMP
  Top 0.254: 48.15,26.62 U8.4
  Top 0.813: C2.1 R25.2 48.15,26.62 | U8.4 50.35,26.74 C28.2
A_MIC_OUT
  Top 0.813: R24.2 40.08,31.93 | 40.08,31.93 C24.1 | U5.2 43.08,34.92 40.08,31.93
ANT
  Bottom 0.32: A2.0 L1.2
AUDIO_OUT  (via drill 0.3)
  Top 0.406: U5.5 47.12,32.38 v46.74,32.77
  Route2 0.254: TP11.TESTPOINT 46.74,43.18
  Route2 0.406: v46.74,32.77 46.74,43.18 46.74,63.25 42.67,67.31 41.15,67.31 40.39,68.07 40.39,79.78 ASSY1.B2
AUDIO_PWR_EN
  Top 0.254: SW3.4 53.74,31.17 R21.1 55.88,32.44 55.88,35.31 53.34,37.85 | ASSY1.B4 46.99,70.99 46.99,44.2 53.34,37.85 | TP10.TESTPOINT 53.34,37.85
AVDD1  (via drill 0.2)
  Top 0.406: v9.88,14.12 10.29,13.72 14.99,13.72 15.75,14.48 17.96,14.48 v19.89,12.55
  Bottom 0.203: U7.35 9.17,12.93 9.09,13.03 9.09,13.23 9.19,13.33 U7.36 9.65,13.89 v9.88,14.12 9.83,14.18 8.88,14.18 C8.1 | L3.1 C22.1 19.84,12.5 v19.89,12.55
BLE_PWR_EN  (via drill 0.3)
  Top 0.254: v20.83,12.19 20.83,25.65 28.57,33.4 | 28.57,33.4 32.77,37.59 43.18,37.59 46.48,40.89 46.48,68.96 ASSY1.B5 | TP9.TESTPOINT 25.4,36.58 28.57,33.4
  Bottom 0.203: SW5.4 18.04,7.62 18.29,7.37 19.3,7.37 21.08,9.14 21.08,11.43 20.65,11.43 R20.1
  Bottom 0.254: 21.08,11.43 21.08,11.94 v20.83,12.19
BLE_RXD  (via drill 0.3)
  Route2 0.254: ASSY1.C3 10.67,65.3 10.67,52.32 | 10.67,52.32 10.67,43.18 11.68,42.16 11.68,41.66 10.67,40.64 10.67,13.46 10.41,13.21 10.41,8.64 v9.65,7.87 | TP16.TESTPOINT 10.67,52.32
  Bottom 0.203: U7.25 v9.65,7.88 v9.65,7.87
BLE_TXD  (via drill 0.3)
  Route2 0.254: ASSY1.C2 10.16,67.33 10.16,52.58 | 10.16,52.58 10.16,15.49 9.14,14.48 9.14,13.72 9.91,12.95 9.91,9.14 8.89,8.13 8.89,7.62 9.65,6.86 v11.68,6.86 v11.69,6.86 | TP15.TESTPOINT 7.37,52.58 10.16,52.58
  Bottom 0.203: U7.22 11.25,7.55 11.28,7.52 11.69,7.11 v11.69,6.86
DCC1
  Bottom 0.203: U7.2 16.33,12.93 17.09,12.17 17.67,12.17 L2.2
GND  (via drill 0.2, 0.3)
  Top 0.254: SW1.2 10.54,42.8 SW1.PAD
  Top 0.813: 10.67,35.05 12.75,37.13 J1.MOUNT0 12.75,38.3 11.18,39.88 | J1.MOUNT3 13.36,24.64 10.67,24.64
  Bottom 0.203: C16.2 16.13,7.37 15.75,7.75 15.23,7.75 U7.13 14.85,8.8 v14.17,9.6 | 8.08,12.53 8.09,12.53 U7.34 10.88,12.53 v11.12,12.65 10.48,12.13 U7.33 | v14.17,11.63 v14.17,12.65 | U7.GND v13.16,11.63
  Bottom 0.254: v5.84,70.36 U6.CENTER
  Bottom 0.305: B1.GND 8.08,12.53
  Bottom 0.406: ASSY1.GND 27.13,50.75 27.18,50.8
  Bottom 0.813: v27.18,91.69 18.03,82.55 13.97,82.55 v10.41,86.11
  other vias: 12.14,11.63 12.14,10.62 12.14,9.6 12.14,12.65 11.13,11.63 11.13,10.62 11.13,9.6 13.16,9.6 13.16,10.62 13.16,12.65 14.17,10.62 38.1,24.38 38.1,25.15 37.39,23.11 37.34,23.88 36.58,24.13 36.07,24.89 36.07,22.61 35.31,23.37 35.31,21.34 39.37,25.15 39.37,24.38 39.37,23.62 39.62,22.86 39.62,22.1 39.12,21.34 38.35,21.34 37.85,20.83 37.85,20.07 37.85,19.3 36.32,19.3 36.32,20.07 36.32,20.83 33.53,24.38 33.78,22.35 22.1,1.27 22.1,3.81 22.1,6.35 22.86,8.89 22.86,11.43 22.86,13.97 1.27,13.97 2.54,13.97 3.81,13.97 5.08,13.97 6.35,13.97 1.27,7.37 2.54,7.37 3.81,7.37 5.08,7.62 6.35,7.37 6.6,8.64 6.6,9.91 46.99,1.27 46.99,3.81 46.99,6.35 46.99,8.89 46.99,11.43 46.99,13.97 46.99,16.51 46.99,19.05 44.45,19.3 41.91,19.3 39.37,19.3 34.8,19.3 32.26,19.3 29.72,19.3 27.18,19.05 39.37,6.35 39.37,8.89 39.37,11.43 38.61,13.97 38.61,3.81 35.56,3.81 35.56,1.27 38.61,1.27 37.08,1.27 37.08,3.81 37.08,6.35 37.08,8.89 37.08,11.43 37.08,13.97 34.8,6.35 34.8,8.89 34.8,11.43 35.56,13.97 32.26,6.35 32.26,8.89 32.26,11.43 29.72,6.35 29.72,8.89 29.72,11.43 41.91,6.35 41.91,8.89 41.91,11.43 44.45,6.35 44.45,8.89 44.45,11.43 27.18,1.27 27.18,3.81 27.18,6.35 27.18,8.89 27.18,11.43 27.18,13.97 27.18,16.51 24.64,1.27 24.64,3.81 24.64,6.35 24.64,8.89 24.64,11.43 24.64,13.97 10.41,87.12 10.41,85.09 7.87,65.28 5.33,72.14 6.86,70.36 6.86,69.34 5.84,69.34 42.16,32.26 43.69,27.18 5.59,39.12 36.07,38.61 52.58,29.72 54.61,33.53 14.73,7.11 19.56,9.65 8.89,19.3 19.81,14.48 19.56,3.81 19.56,1.27 6.35,1.27 3.81,1.27 1.27,1.27 1.27,3.81 1.27,6.35 3.05,3.05 7.37,6.35 7.37,7.62 1.27,16.51 3.81,16.51 6.1,16.51 1.27,19.05 3.81,19.05 6.35,19.05 8.89,21.34 43.94,70.1 44.7,69.34 45.47,68.58 43.94,67.82 44.7,67.06 45.47,66.29 46.48,72.64 45.72,73.41 43.94,75.18 44.2,72.64 44.96,71.88 45.72,71.12 49.53,1.27 49.53,3.81 49.53,6.35 49.53,8.89 52.07,8.89 54.61,1.27 54.61,3.81 54.61,6.35 52.07,19.05 52.07,16.51 52.07,21.59 49.53,13.97 49.53,11.43 52.07,13.97 52.07,11.43 55.63,12.7 55.63,19.05 55.63,16.51 55.63,21.59 27.18,21.59 29.72,21.59 32.26,21.59 32.26,24.13 29.72,24.13 27.18,24.13 27.18,26.67 29.72,26.67 29.72,29.21 27.18,29.21 32.26,29.21 34.8,29.21 37.34,29.21 34.8,31.75 32.26,31.75 32.26,34.29 34.8,34.29 37.34,34.29 41.91,21.59 49.53,19.05 48.26,17.78 49.53,21.59 29.72,31.75 28.7,34.54 26.92,33.78 43.94,64.77 44.7,64.01 45.47,63.25 2.79,65.02
  pour Top (rank 2): 57.15,-3.05 0,-3.05 0,92.96 57.15,92.96
  pour Route2 (rank 2): 57.15,-2.03 0,-2.03 0,92.96 57.15,92.96
  pour Bottom (rank 3): 57.15,0 0,0 0,92.96 57.15,92.96
  pour Bottom (rank 2, no thermals): 2.29,7.37 2.29,9.4 0.76,9.4 0.76,7.37
GND2  (via drill 0.3)
  other vias: 52.07,1.27
GPS_PWR_EN  (via drill 0.3)
  Top 0.254: v37.08,49.02 37.08,50.42 ASSY1.D3 20.02,63.45 TP22.TESTPOINT
  Bottom 0.254: SW2.4 37.52,46.37 R18.1 37.52,48.59 v37.08,49.02
GPS_RF_IN
  Bottom 0.32: U2.4 38.74,26.36 U4.11
GPS_RXD
  Bottom 0.254: L5.2 33.27,46.48 36.58,49.78 40.26,49.78 ASSY1.TX 44.65,48.21 TP1.TESTPOINT
GPS_TXD
  Bottom 0.254: ASSY1.RX 37.03,50.75 32,45.72 32,39.12 | L4.2 32,39.12 | TP2.TESTPOINT 30.48,39.12 32,39.12
GPS_VCC
  Bottom 0.254: R4.2 36.25,42.93 38.02,42.93 | 37.51,36.32 U4.7 | U4.8 38.53,36.06
  Bottom 0.406: 36.83,37.34 37.59,37.34 | 37.59,37.34 38.35,37.34 | 38.35,37.34 38.61,37.08 | 37.59,37.34 37.51,37.25 | 38.35,37.34 38.53,37.52 C15.2 | SW2.1 37.78,44.74 | U4.6 36.41,36.91
  Bottom 0.61: 38.53,36.06 C15.2 C27.2 38.53,41.66 C12.2 38.02,42.93 38.02,44.5 37.78,44.74 | 38.35,37.34 36.83,37.34 36.41,36.91 | 37.51,37.25 37.51,36.32
LED
  Top 0.254: ASSY1.C5 14.13,63.69 D3.C
LNA_IN
  Bottom 0.254: 37.08,21.13 U1.5
  Bottom 0.32: L1.1 37.08,21.13
LNA_OUT
  Bottom 0.254: 37.59,22.09 U1.3
  Bottom 0.305: U2.1 38.44,22.09
  Bottom 0.32: 38.44,22.09 37.59,22.09
N$1
  Bottom 0.254: D1.A 34.54,42.09 R4.1
N$2
  Bottom 0.254: U4.4 34.21,38.03 D1.C
N$3
  Top 0.254: D3.A 15.42,55.92 R6.2
N$4
  Top 0.813: MK1.TERM+ 53.22,26.62 C28.1 53.87,26.02 R7.1
N$5
  Top 0.254: 46.85,27.83 46.85,27.69
  Top 0.406: 46.85,27.83 46.04,28.64 U8.1 45.37,28.7 R1.2 | 46.85,27.69 R25.1
  Top 0.813: C2.2 R25.1
N$6
  Top 0.406: C7.2 49.78,36.37 U5.8
N$7
  Top 0.406: R1.1 40.51,28.7 C24.2
N$8  (via drill 0.3)
  other vias: 6.35,21.34
N$9
  Top 0.813: U8.3 44.58,25.88 C23.2 42.2,24.57 R23.2 42.31,24.67 R22.1
N$10
  Bottom 0.203: B1.ANT1 8.74,11.33 U7.31
N$11
  Top 0.406: U5.6 47.62,33.66 45.09,36.2 U5.1 42.22,36.2 C21.1
N$12
  Bottom 0.203: B1.ANT2 8.74,11.73 U7.32
N$13
  Bottom 0.254: C1.1 6.81,11.78
  Bottom 0.305: C1.1 6.6,11.78 1.52,11.78 A1.S1
  Bottom 0.32: B1.SE 6.86,11.53 6.6,11.78
N$14
  Bottom 0.254: SW4.1 8.38,83.56 7.62,82.8 | ASSY2.8 5.08,82.8 7.62,82.8 | 7.62,82.8 ASSY2.4
N$15
  Bottom 0.203: L2.1 18.96,10.63 L3.2
N$16  (via drill 0.3)
  other vias: 3.81,21.34
N$17  (via drill 0.3)
  other vias: 1.27,21.34
N$18
  Top 0.254: R16.2 1.6,40.64
  Top 0.406: SW1.1 10.03,43.26 9.67,43.26 8.64,42.23 R12.2 | R13.2 R12.2 | R12.2 7.87,41.33 | 7.87,41.33 7.47,41.33 7.29,41.15 | 7.29,41.15 C26.1 | R14.2 2.87,40.72 | 2.87,40.72 3.3,41.15 7.29,41.15 | R16.2 2.72,40.56 2.87,40.72 | J1.4 7.87,38.03 7.87,40.89 7.87,41.33
N$20
  Bottom 0.203: U7.37 10.45,14.49 10.24,14.71 8.71,14.71 8.33,15.09 8.33,15.8 X2.1 8.33,15.8 C3.1
N$21
  Bottom 0.203: X2.3 9.99,16.79 C4.1 10.85,16.63 10.62,16.4 10.62,14.83 10.85,14.6 U7.38
N$22
  Bottom 0.203: C9.1 11.25,14.99 11.25,14.73 U7.39
N$24
  Bottom 0.203: U7.29 9.21,10.53 8.69,10.01 C14.1
N$25
  Bottom 0.203: D2.A 17.7,15.64 R5.2
N$26
  Bottom 0.203: S1.2 14.36,4.88 R2.2
N$33
  cutout Bottom: 26.16,92.96 11.18,92.96 11.18,18.8 16.76,18.8 16.76,15.24 26.16,15.24
  cutout Route15: 26.16,92.96 11.18,92.96 11.18,15.24 26.16,15.24 26.16,41.66 22.86,41.66 22.86,44.45 26.16,44.45
  cutout Route2: 26.16,92.96 11.18,92.96 11.18,15.24 26.16,15.24
  cutout Top: 26.16,92.96 11.18,92.96 11.18,15.24 26.16,15.24
N$34
  cutout Bottom: 6.1,10.67 9.91,10.67 9.91,12.45 6.1,12.45 6.1,13.21 0,13.21 0,8.13 0.76,8.13 0.76,9.4 2.29,9.4 2.29,8.13 6.1,8.13
N$37
  cutout Top: 0,13.21 6.1,13.21 6.1,8.13 0,8.13
N$40
  Bottom 0.254: U4.2 L4.1
N$41
  Bottom 0.254: L5.1 33.27,36.16 U4.3
NRF_A2
  Bottom 0.203: 14.24,17.32 X1.B | X1.B 14.05,17.21 U7.46 | X1.B 14.68,17.14 C6.1
NRF_A3
  Bottom 0.203: U7.45 13.65,16.94 X1.A 12.65,17.04 C5.1
NRF_P29
  Bottom 0.203: U7.48 15.7,14.98 15.7,16.48 17.36,18.15 D2.C
NRF_SWDCLK
  Bottom 0.203: U7.24 10.45,7.56 R15.1 10.45,4.2 J2.4
NRF_SWDIO/!RESET
  Bottom 0.203: J2.2 10.97,4.95 10.97,5.31 | 10.97,5.31 10.97,7.4 10.85,7.52 U7.23 | R2.1 11.01,5.34 10.97,5.31
  Bottom 0.254: R2.1 13.03,5.66 13.21,5.84 18.29,5.84 21.59,9.14 21.59,32.26 | 21.59,32.26 21.59,50.83 ASSY1.D7 | 21.59,32.26 TP25.TESTPOINT
REGOUT
  Bottom 0.254: C18.1 6.17,66.47 6.15,66.49 U6.10
SD_ENABLE_POWER
  Top 0.254: SW1.4 11.73,43.51 R17.1
SD_MISO  (via drill 0.3)
  Top 0.254: J1.7 4.57,38.03 v4.57,39.12 4.57,39.3 R14.1
  Route2 0.254: ASSY1.A4 42.14,61.21 TP4.TESTPOINT
  Bottom 0.254: v4.57,39.12 5.33,39.88 5.84,39.88 6.43,39.29 7.8,39.29 8.13,39.62 8.13,40.64 22.86,55.37 22.86,56.64 23.37,57.15 38.08,57.15 ASSY1.A4
SD_MOSI  (via drill 0.3)
  Top 0.254: R12.1 8.89,40.21 v8.89,39.37 8.89,38.11 J1.3
  Bottom 0.254: v8.89,39.37 10.16,40.64 10.16,42.16 14.73,46.74 | ASSY1.A5 38.08,54.61 22.61,54.61 14.73,46.74 | TP3.TESTPOINT 14.73,46.74
SD_SCLK  (via drill 0.3)
  Top 0.254: J1.5 6.8,39.57 v7.11,39.88
  Bottom 0.254: ASSY1.A3 38.08,59.69 23.37,59.69 22.35,58.67 22.35,55.37 14.1,47.11 | v7.11,39.88 7.11,40.13 14.1,47.11 | TP5.TESTPOINT 14.1,47.11
SENSORS_SCL  (via drill 0.3)
  Top 0.254: v39.12,42.42 39.12,53.47 ASSY1.D1 | v7.87,73.41 8.13,73.41 v9.14,72.39
  Bottom 0.254: U6.23 R10.1 7.67,73.2 v7.87,73.41 | v9.14,72.39 18.54,72.39 | 18.54,72.39 20.19,72.39 ASSY1.D1 | U3.5 51.25,35.07 50.98,35.07 44.9,41.15 40.39,41.15 v39.12,42.42 | TP20.TESTPOINT 18.54,72.39
SENSORS_SDA  (via drill 0.3)
  Top 0.254: v40.13,42.42 40.13,54.99 ASSY1.D0
  Bottom 0.254: U6.24 7.35,71.86 R9.1 | R9.1 8.89,73.41 | ASSY1.D0 21.87,73.25 10.67,73.25 | 10.67,73.25 R9.1 | U3.6 45.16,41.66 40.89,41.66 v40.13,42.42 | 10.67,73.25 10.67,74.17 9.91,74.93 5.59,74.93 1.91,71.25 1.78,71.12 1.02,70.36 1.02,54.1 TP19.TESTPOINT 1.78,53.34
VCC  (via drill 0.3)
  Top 0.254: SW1.3 11.68,42.65 R17.2 12.02,41.91 v10.92,41.91 | R6.1 14.3,54.36 v8.38,54.36 | SW3.3 53.74,30.3 R21.2 53.77,29.46 v53.59,29.46
  Top 0.406: R17.2 23.57,42.65 ASSY1.3V3
  Route15 0.813: 27.18,89.92 25.4,89.92 18.03,82.55 13.97,82.55 12.45,84.07 10.41,84.07
  Bottom 0.203: v19.56,8.64 20.57,9.65 R20.2
  Bottom 0.254: 52.83,35.42 U3.1 54.04,35.42 C17.1 54.1,35.81 v53.59,36.32 | U6.13 3.5,68.85 C19.1 3.48,68.25 2.62,67.39 R11.2 | U6.8 6.95,67.8 C13.1 7.7,66.47 v7.87,66.29 | U6.22 6.55,71.94 5.21,73.28 | U6.1 8.64,71.59 v8.64,71.63 | R3.1 55.09,8.64 v54.1,8.64 | R8.2 41.68,39.12 40.92,39.88 v40.89,39.88 | SW5.3 18.83,7.91 v19.56,8.64 | SW4.3 7.88,86.03 | 7.88,86.03 R19.2 | v7.37,86.36 7.69,86.03 7.88,86.03
  Bottom 0.406: 3.5,68.85 3.5,71.57 v4.06,72.14 5.21,73.28 6,74.07 R10.2 7.01,74.12 R9.2 | SW2.3 36.65,46.37 R18.2 v35.81,47.24
  pour Route15 (rank 2): 57.15,-1.02 0,-1.02 0,92.96 57.15,92.96
VCC_A_MIC
  Top 0.406: C20.1 43.36,30.66 42.93,30.23 41.4,30.23 41.15,30.48 39.12,30.48 38.61,29.97 38.61,27.69 40.13,26.16 R22.2 | SW3.1 51.28,30.99
  Top 0.813: C20.1 44.45,30.99 | 44.45,30.99 48.01,30.99 | 51.28,30.99 48.01,30.99 | U5.7 50.8,34.92 51.56,34.16 51.56,31.27 51.28,30.99 | U8.5 48.04,30.96 48.01,30.99 | U5.4 44.37,31.06 44.45,30.99 | R7.2 54.75,28.45 52.58,28.45 51.28,29.74 51.28,30.99
VCC_BLE  (via drill 0.3)
  Top 0.406: v16.51,13.72 v16.51,9.14 16.51,4.83 v12.95,1.27
  Bottom 0.203: 15.76,8.93 U7.12 15.78,8.93 16.16,8.55 16.16,8.38 C16.1 | 17.1,13.33 C25.1
  Bottom 0.254: U7.1 16.13,13.33 v16.51,13.72 16.28,13.95 R5.1
  Bottom 0.406: 16.16,8.38 16.51,8.73 v16.51,9.14 16.73,9.36 SW5.1 | C25.1 16.93,13.72 v16.51,13.72 | v12.95,1.27 11.73,2.49 J2.1
VCC_RF
  Bottom 0.203: U1.2 37.08,22.61 35.31,24.38 C11.2 | U1.6 36.59,21.59 36.58,21.59
  Bottom 0.254: C11.2 35.31,24.46
  Bottom 0.32: 35.31,24.46 U4.14 | 36.58,21.59 36.07,21.59 34.54,23.11 34.54,23.62 35.23,24.31 C11.2
VDD_PA1
  Bottom 0.203: U7.30 9,10.93 8.54,10.47 C10.1 8.09,11.27 B1.VCC
WIFI_PWR_EN
  Bottom 0.254: SW4.4 9.07,86 R19.1 9.83,85.6 9.83,84.85 12.89,81.79 22.1,81.79 22.86,82.55 40.62,82.55 ASSY1.B1 45.47,87.4 TP12.TESTPOINT
WIFI_RXD
  Top 0.254: ASSY1.C1 20.55,80.26 18.29,80.26 | ASSY2.7 5.08,80.26 18.29,80.26 | TP14.TESTPOINT 18.29,80.26
WIFI_TXD
  Top 0.254: ASSY1.C0 19.28,81.53 ASSY2.2 8.38,84.58 TP13.TESTPOINT

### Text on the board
tNames: WIFI_PWR_EN | WIFI_TXD | WIFI_RXD | !WIFI_RESET | Noah Klugman / Branden Ghena / Neal Jackson / 01/18 | SENSORS_SCL | GPS_PWR_EN | SD_MISO | !GPS_RESET | !SAFEMODE | !IMU_INT | SENSE_SDA | BLE_TXD | BLE_RXD | !LIGHT_INT | GPS_RXD | SD_SCLK | SD_MOSI | AUDIO_OUT | !SD_CS | GPS_TXD | AUDIO_PWR_EN | BLE_PWR_EN | SD_DETECT | NRF_SWDIO/!RESET
bNames: RESET
Document: Antenna Entry / (from below) | Cell Antenna below / (No solid groundplane) | Wire Entry (above board)

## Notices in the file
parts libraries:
SparkFun-Aesthetics: Licensing: Creative Commons ShareAlike 4.0 International - https://creativecommons.org/licenses/by-sa/4.0
